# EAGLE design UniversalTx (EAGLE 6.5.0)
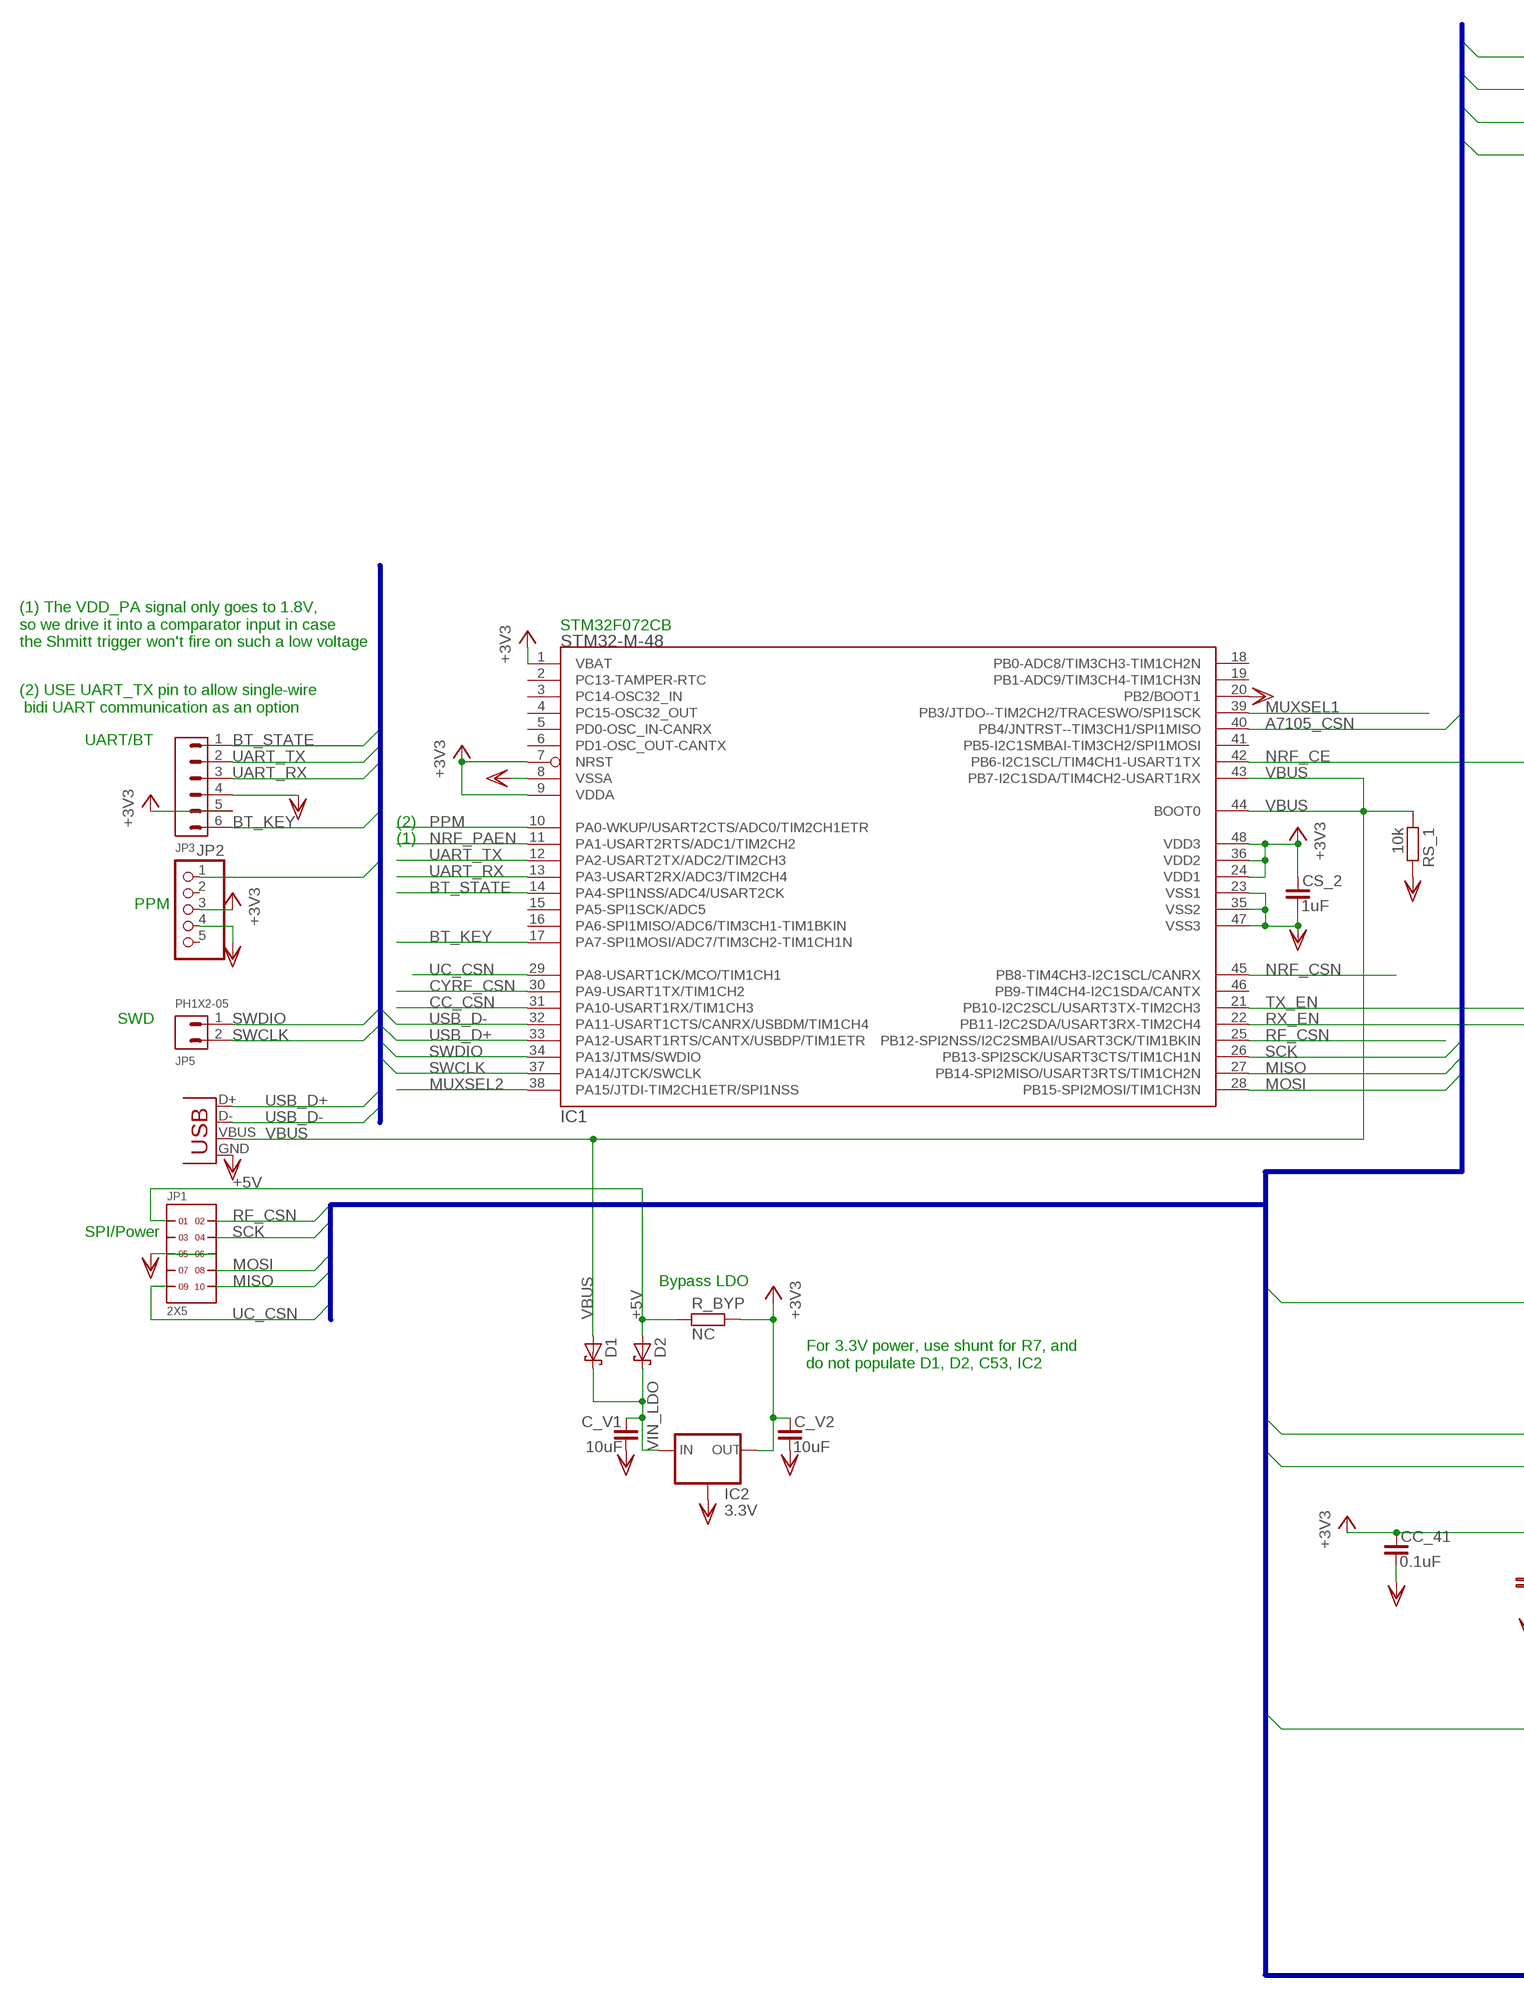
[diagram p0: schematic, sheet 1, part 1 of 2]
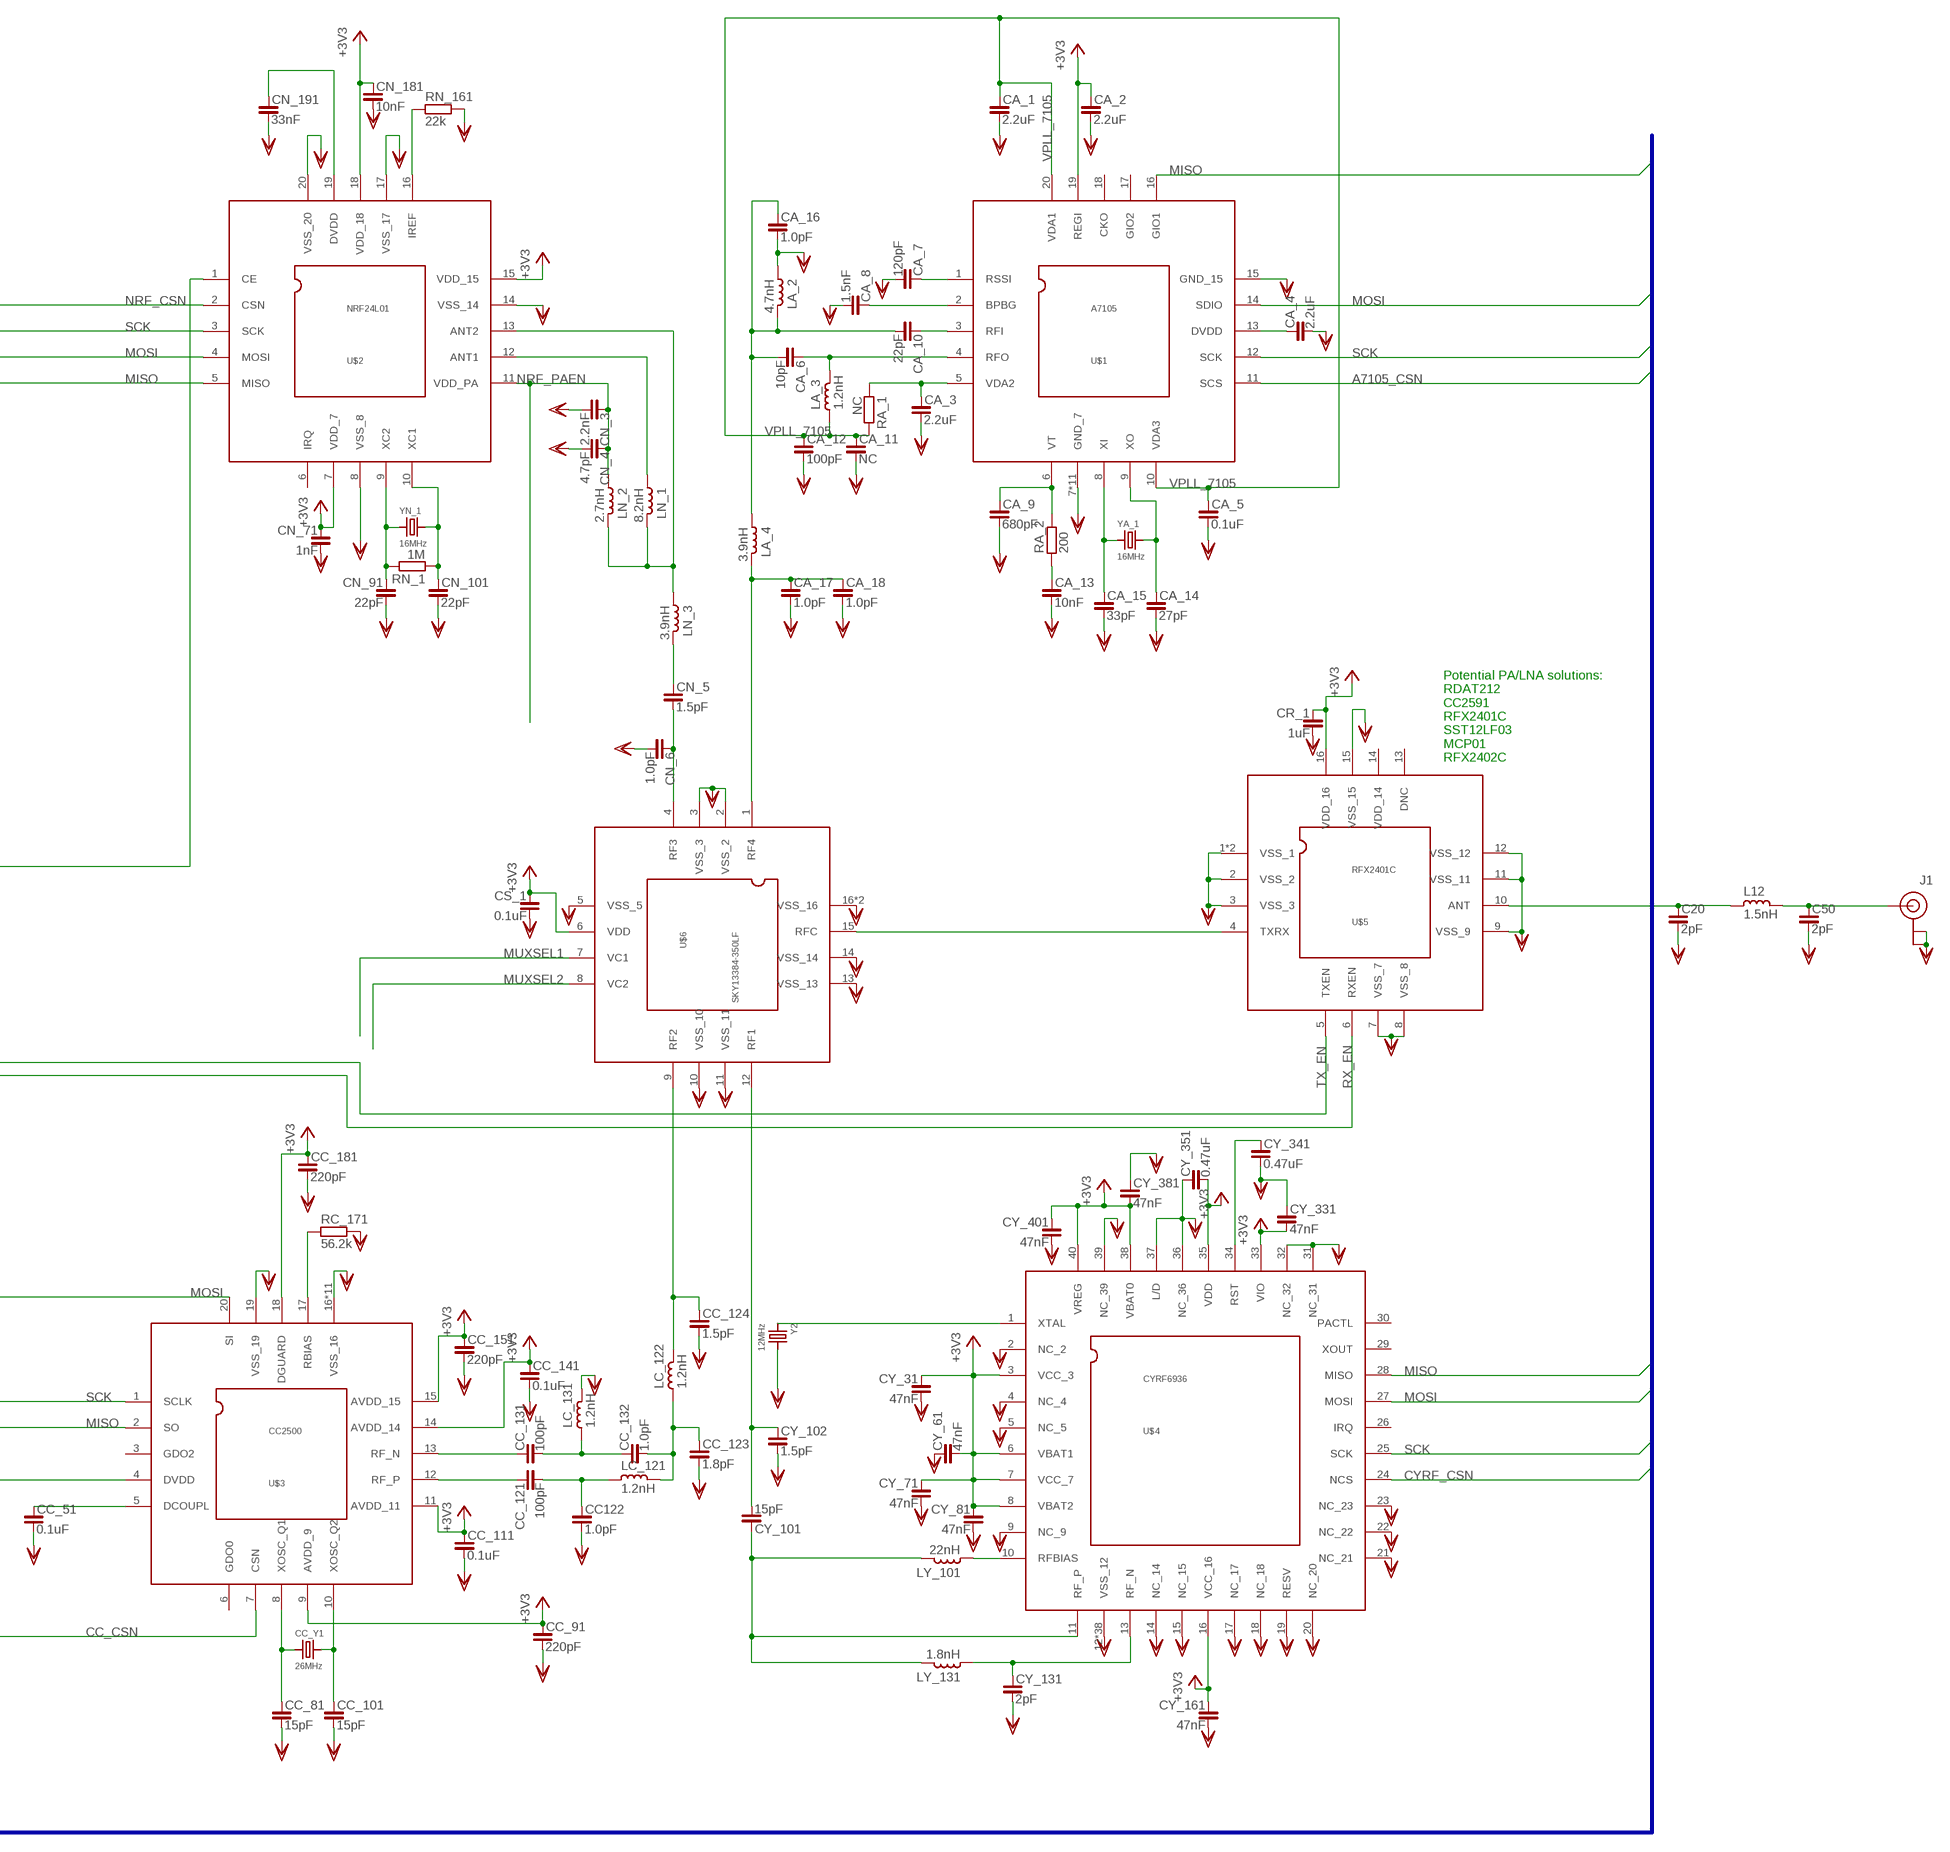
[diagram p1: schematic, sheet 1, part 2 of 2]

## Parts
C20  2pF  C_0402  [C0402]
C50  2pF  C_0402  [C0402]
C_V1  10uF  C_0805  [C0805]
C_V2  10uF  C_0805  [C0805]
CA_1  2.2uF  C_0402  [C0402]
CA_2  2.2uF  C_0402  [C0402]
CA_3  2.2uF  C_0402  [C0402]
CA_4  2.2uF  C_0402  [C0402]
CA_5  0.1uF  C_0402  [C0402]
CA_6  10pF  C_0402  [C0402]
CA_7  120pF  C_0402  [C0402]
CA_8  1.5nF  C_0402  [C0402]
CA_9  680pF  C_0402  [C0402]
CA_10  22pF  C_0402  [C0402]
CA_11  NC  C_0402  [C0402]
CA_12  100pF  C_0402  [C0402]
CA_13  10nF  C_0402  [C0402]
CA_14  27pF  C_0402  [C0402]
CA_15  33pF  C_0402  [C0402]
CA_16  1.0pF  C_0402  [C0402]
CA_17  1.0pF  C_0402  [C0402]
CA_18  1.0pF  C_0402  [C0402]
CC122  1.0pF  C_0402  [C0402]
CC_41  0.1uF  C_0402  [C0402]
CC_51  0.1uF  C_0402  [C0402]
CC_81  15pF  C_0402  [C0402]
CC_91  220pF  C_0402  [C0402]
CC_101  15pF  C_0402  [C0402]
CC_111  0.1uF  C_0402  [C0402]
CC_121  100pF  C_0402  [C0402]
CC_123  1.8pF  C_0402  [C0402]
CC_124  1.5pF  C_0402  [C0402]
CC_131  100pF  C_0402  [C0402]
CC_132  1.0pF  C_0402  [C0402]
CC_141  0.1uF  C_0402  [C0402]
CC_151  220pF  C_0402  [C0402]
CC_181  220pF  C_0402  [C0402]
CC_Y1  26MHz  CRYSTAL.3.2X2.5MM  [3.2X2.5MM]
CN_3  2.2nF  C_0402  [C0402]
CN_4  4.7pF  C_0402  [C0402]
CN_5  1.5pF  C_0402  [C0402]
CN_6  1.0pF  C_0402  [C0402]
CN_71  1nF  C_0402  [C0402]
CN_91  22pF  C_0402  [C0402]
CN_101  22pF  C_0402  [C0402]
CN_181  10nF  C_0402  [C0402]
CN_191  33nF  C_0402  [C0402]
CR_1  1uF  C_0402  [C0402]
CS_1  0.1uF  C_0402  [C0402]
CS_2  1uF  C_0402  [C0402]
CY_31  47nF  C_0402  [C0402]
CY_61  47nF  C_0402  [C0402]
CY_71  47nF  C_0402  [C0402]
CY_81  47nF  C_0402  [C0402]
CY_101  15pF  C_0402  [C0402]
CY_102  1.5pF  C_0402  [C0402]
CY_131  2pF  C_0402  [C0402]
CY_161  47nF  C_0402  [C0402]
CY_331  47nF  C_0402  [C0402]
CY_341  0.47uF  C_0402  [C0402]
CY_351  0.47uF  C_0402  [C0402]
CY_381  47nF  C_0402  [C0402]
CY_401  47nF  C_0402  [C0402]
D1  LSM115J  [DO214BA]
D2  LSM115J  [DO214BA]
IC1  STM32-M-48  [LQFP48]
IC2  3.3V  LD1117SOT223  [SOT223]
J1  U.FL  [U.FL]
JP1  2X5  [2X5]
JP2  PINHD-1X05_2.54-S  [1X05-S]
JP3  PH1X6-05  [PH005-1-6]
JP5  PH1X2-05  [PH005-1-2]
JP6  USBSMD  [USB-MINIB]
L12  1.5nH  L_0402  [L0402]
LA_2  4.7nH  L_0402  [L0402]
LA_3  1.2nH  L_0402  [L0402]
LA_4  3.9nH  L_0402  [L0402]
LC_121  1.2nH  L_0402  [L0402]
LC_122  1.2nH  L_0402  [L0402]
LC_131  1.2nH  L_0402  [L0402]
LN_1  8.2nH  L_0402  [L0402]
LN_2  2.7nH  L_0402  [L0402]
LN_3  3.9nH  L_0402  [L0402]
LY_101  22nH  L_0402  [L0402]
LY_131  1.8nH  L_0402  [L0402]
R_BYP  NC  R_0805  [R0805]
RA_1  NC  R_0402  [R0402]
RA_2  200  R_0402  [R0402]
RC_171  56.2k  R_0402  [R0402]
RN_1  1M  R_0402  [R0402]
RN_161  22k  R_0402  [R0402]
RS_1  10k  R_0402  [R0402]
U$1  A7105  [QFN20-4X4-PAD]
U$2  NRF24L01  [QFN20-4X4-NRF]
U$3  CC2500  [QFN20-4X4-PAD]
U$4  CYRF6936  [QFN40-6X6]
U$5  RFX2401C  [QFN16-3X3-PAD]
U$6  SKY13384-350LF  [QFN16-3X3-PAD]
Y2  12MHz  CRYSTAL.3.2X2.5MM  [3.2X2.5MM]
YA_1  16MHz  CRYSTAL.3.2X2.5MM  [3.2X2.5MM]
YN_1  16MHz  CRYSTAL.3.2X2.5MM  [3.2X2.5MM]

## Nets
+3V3: C_V2.1 CA_2.1 CC_41.1 CC_91.1 CC_111.1 CC_141.1 CC_151.1 CC_181.1 CN_71.1 CN_181.1 CR_1.1 CS_1.1 CS_2.1 CY_31.1 CY_61.2 CY_71.1 CY_81.1 CY_161.1 CY_331.2 CY_351.2 CY_381.2 CY_401.1 IC1.1(VBAT) IC1.7(NRST) IC1.9(VDDA) IC1.24(VDD1) IC1.36(VDD2) IC1.48(VDD3) IC2.2(OUT) JP2.3 JP3.5 R_BYP.2 U$1.19(REGI) U$2.7(VDD_7) U$2.15(VDD_15) U$2.18(VDD_18) U$3.4(DVDD) U$3.9(AVDD_9) U$3.11(AVDD_11) U$3.14(AVDD_14) U$3.15(AVDD_15) U$3.18(DGUARD) U$4.3(VCC_3) U$4.6(VBAT1) U$4.7(VCC_7) U$4.8(VBAT2) U$4.16(VCC_16) U$4.33(VIO) U$4.35(VDD) U$4.38(VBAT0) U$4.40(VREG) U$5.16(VDD_16) U$6.6(VDD)
+5V: D2.A JP1.1 R_BYP.1
A7105_CSN: IC1.40(PB4/JNTRST--TIM3CH1/SPI1MISO) U$1.11(SCS)
BT_KEY: IC1.17(PA7-SPI1MOSI/ADC7/TIM3CH2-TIM1CH1N) JP3.6
BT_STATE: IC1.14(PA4-SPI1NSS/ADC4/USART2CK) JP3.1
CC_CSN: IC1.31(PA10-USART1RX/TIM1CH3) U$3.7(CSN)
CYRF_CSN: IC1.30(PA9-USART1TX/TIM1CH2) U$4.24(NCS)
MISO: IC1.27(PB14-SPI2MISO/USART3RTS/TIM1CH2N) JP1.10 U$1.16(GIO1) U$2.5(MISO) U$3.2(SO) U$4.28(MISO)
MOSI: IC1.28(PB15-SPI2MOSI/TIM1CH3N) JP1.8 U$1.14(SDIO) U$2.4(MOSI) U$3.20(SI) U$4.27(MOSI)
MUXSEL1: IC1.39(PB3/JTDO--TIM2CH2/TRACESWO/SPI1SCK) U$6.7(VC1)
MUXSEL2: IC1.38(PA15/JTDI-TIM2CH1ETR/SPI1NSS) U$6.8(VC2)
N$1: CN_101.1 RN_1.1 U$2.10(XC1) YN_1.3
N$2: CN_91.1 RN_1.2 U$2.9(XC2) YN_1.1
N$3: CN_191.1 U$2.19(DVDD)
N$4: CA_9.1 RA_2.2 U$1.6(VT)
N$5: LN_1.1 LN_2.1 LN_3.2 U$2.13(ANT2)
N$7: C50.1 J1.P$3(SIGNAL) L12.1
N$8: CN_5.1 LN_3.1
N$9: CN_5.2 CN_6.1 U$6.4(RF3)
N$10: RN_161.1 U$2.16(IREF)
N$11: CA_13.1 RA_2.1
N$12: CA_14.1 U$1.9(XO) YA_1.3
N$14: CC_131.1 U$3.13(RF_N)
N$15: LN_1.2 U$2.12(ANT1)
N$16: CC_121.1 U$3.12(RF_P)
N$17: CA_15.1 U$1.8(XI) YA_1.1
N$18: CA_4.1 U$1.13(DVDD)
N$24: CC_123.1 CC_132.2 LC_121.1 LC_122.2
N$25: CA_17.1 CA_18.1 LA_4.1 U$6.1(RF4)
N$26: CA_7.1 U$1.1(RSSI)
N$27: CA_8.1 U$1.2(BPBG)
N$28: CA_10.1 U$1.3(RFI)
N$29: CA_6.1 LA_3.1 U$1.4(RFO)
N$30: CA_3.1 RA_1.1 U$1.5(VDA2)
N$31: C20.1 L12.2 U$5.10(ANT)
N$32: CC_51.1 U$3.5(DCOUPL)
N$37: RC_171.1 U$3.17(RBIAS)
N$38: CC_101.1 CC_Y1.3 U$3.10(XOSC_Q2)
N$39: CC_81.1 CC_Y1.1 U$3.8(XOSC_Q1)
N$40: CC122.1 CC_121.2 LC_121.2
N$41: CC_131.2 CC_132.1 LC_131.2
N$42: U$5.4(TXRX) U$6.15(RFC)
N$43: CY_341.1 U$4.34(RST)
N$44: U$4.1(XTAL) Y2.1
N$45: LY_101.2 U$4.10(RFBIAS)
N$46: CY_101.1 LY_101.1 LY_131.1 U$4.11(RF_P)
N$47: CY_131.1 LY_131.2 U$4.13(RF_N)
N$48: CA_6.2 CA_10.2 CA_16.1 LA_2.1 LA_4.2
N$49: CY_101.2 CY_102.1 U$6.12(RF1)
N$50: CC_124.1 LC_122.1 U$6.9(RF2)
NRF_CE: IC1.42(PB6-I2C1SCL/TIM4CH1-USART1TX) U$2.1(CE)
NRF_CSN: IC1.45(PB8-TIM4CH3-I2C1SCL/CANRX) U$2.2(CSN)
NRF_PAEN: CN_3.1 CN_4.1 IC1.11(PA1-USART2RTS/ADC1/TIM2CH2) LN_2.2 U$2.11(VDD_PA)
PPM: IC1.10(PA0-WKUP/USART2CTS/ADC0/TIM2CH1ETR) JP2.1
RF_CSN: IC1.25(PB12-SPI2NSS/I2C2SMBAI/USART3CK/TIM1BKIN) JP1.2
RX_EN: IC1.22(PB11-I2C2SDA/USART3RX-TIM2CH4) U$5.6(RXEN)
SCK: IC1.26(PB13-SPI2SCK/USART3CTS/TIM1CH1N) JP1.4 U$1.12(SCK) U$2.3(SCK) U$3.1(SCLK) U$4.25(SCK)
SWCLK: IC1.37(PA14/JTCK/SWCLK) JP5.2
SWDIO: IC1.34(PA13/JTMS/SWDIO) JP5.1
TX_EN: IC1.21(PB10-I2C2SCL/USART3TX-TIM2CH3) U$5.5(TXEN)
UART_RX: IC1.13(PA3-USART2RX/ADC3/TIM2CH4) JP3.3
UART_TX: IC1.12(PA2-USART2TX/ADC2/TIM2CH3) JP3.2
UC_CSN: IC1.29(PA8-USART1CK/MCO/TIM1CH1) JP1.9
USB_D+: IC1.33(PA12-USART1RTS/CANTX/USBDP/TIM1ETR) JP6.D+
USB_D-: IC1.32(PA11-USART1CTS/CANRX/USBDM/TIM1CH4) JP6.D-
VBUS: D1.A IC1.43(PB7-I2C1SDA/TIM4CH2-USART1RX) IC1.44(BOOT0) JP6.VBUS RS_1.1
VIN_LDO: C_V1.1 D1.C D2.C IC2.3(IN)
VPLL_7105: CA_1.1 CA_5.1 CA_11.1 CA_12.1 LA_3.2 RA_1.2 U$1.10(VDA3) U$1.20(VDA1)
VSS: C20.2 C50.2 C_V1.2 C_V2.2 CA_1.2 CA_2.2 CA_3.2 CA_4.2 CA_5.2 CA_7.2 CA_8.2 CA_9.2 CA_11.2 CA_12.2 CA_13.2 CA_14.2 CA_15.2 CA_16.2 CA_17.2 CA_18.2 CC122.2 CC_41.2 CC_51.2 CC_81.2 CC_91.2 CC_101.2 CC_111.2 CC_123.2 CC_124.2 CC_141.2 CC_151.2 CC_181.2 CN_3.2 CN_4.2 CN_6.2 CN_71.2 CN_91.2 CN_101.2 CN_181.2 CN_191.2 CR_1.2 CS_1.2 CS_2.2 CY_31.2 CY_61.1 CY_71.2 CY_81.2 CY_102.2 CY_131.2 CY_161.2 CY_331.1 CY_341.2 CY_351.1 CY_381.1 CY_401.2 IC1.8(VSSA) IC1.20(PB2/BOOT1) IC1.23(VSS1) IC1.35(VSS2) IC1.47(VSS3) IC2.1(GND) IC2.4(GND) J1.P$1(GND) J1.P$2(GND) JP1.5 JP1.6 JP2.4 JP3.4 JP6.GND LA_2.2 LC_131.1 RC_171.2 RN_161.2 RS_1.2 U$1.7(GND_7) U$1.15(GND_15) U$1.21(GND_7) U$1.P$1(GND_7) U$1.P$2(GND_7) U$1.P$3(GND_7) U$1.P$4(GND_7) U$1.P$5(GND_7) U$1.P$6(GND_7) U$1.P$7(GND_7) U$1.P$8(GND_7) U$1.P$9(GND_7) U$2.8(VSS_8) U$2.14(VSS_14) U$2.17(VSS_17) U$2.20(VSS_20) U$3.16(VSS_16) U$3.19(VSS_19) U$3.21(VSS_16) U$3.P$1(VSS_16) U$3.P$2(VSS_16) U$3.P$3(VSS_16) U$3.P$4(VSS_16) U$3.P$5(VSS_16) U$3.P$6(VSS_16) U$3.P$7(VSS_16) U$3.P$8(VSS_16) U$3.P$9(VSS_16) U$4.2(NC_2) U$4.4(NC_4) U$4.5(NC_5) U$4.9(NC_9) U$4.12(VSS_12) U$4.14(NC_14) U$4.15(NC_15) U$4.17(NC_17) U$4.18(NC_18) U$4.19(RESV) U$4.20(NC_20) U$4.21(NC_21) U$4.22(NC_22) U$4.23(NC_23) U$4.31(NC_31) U$4.32(NC_32) U$4.36(NC_36) U$4.37(L/D) U$4.39(NC_39) U$4.P$1(VSS_12) U$4.P$2(VSS_12) U$4.P$3(VSS_12) U$4.P$4(VSS_12) U$4.P$5(VSS_12) U$4.P$6(VSS_12) U$4.P$7(VSS_12) U$4.P$8(VSS_12) U$4.P$9(VSS_12) U$4.P$10(VSS_12) U$4.P$11(VSS_12) U$4.P$12(VSS_12) U$4.P$13(VSS_12) U$4.P$14(VSS_12) U$4.P$15(VSS_12) U$4.P$16(VSS_12) U$4.P$17(VSS_12) U$4.P$18(VSS_12) U$4.P$19(VSS_12) U$4.P$20(VSS_12) U$4.P$21(VSS_12) U$4.P$22(VSS_12) U$4.P$23(VSS_12) U$4.P$24(VSS_12) U$4.P$25(VSS_12) U$4.P$26(VSS_12) U$4.P$27(VSS_12) U$4.P$28(VSS_12) U$4.P$29(VSS_12) U$4.P$30(VSS_12) U$4.P$31(VSS_12) U$4.P$32(VSS_12) U$4.P$33(VSS_12) U$4.P$34(VSS_12) U$4.P$35(VSS_12) U$4.P$36(VSS_12) U$4.P$37(VSS_12) U$5.1(VSS_1) U$5.2(VSS_2) U$5.3(VSS_3) U$5.7(VSS_7) U$5.8(VSS_8) U$5.9(VSS_9) U$5.11(VSS_11) U$5.12(VSS_12) U$5.15(VSS_15) U$5.17(VSS_1) U$6.2(VSS_2) U$6.3(VSS_3) U$6.5(VSS_5) U$6.10(VSS_10) U$6.11(VSS_11) U$6.13(VSS_13) U$6.14(VSS_14) U$6.16(VSS_16) U$6.17(VSS_16) Y2.3
Unconnected: IC1.2(PC13-TAMPER-RTC) IC1.3(PC14-OSC32_IN) IC1.4(PC15-OSC32_OUT) IC1.5(PD0-OSC_IN-CANRX) IC1.6(PD1-OSC_OUT-CANTX) IC1.15(PA5-SPI1SCK/ADC5) IC1.16(PA6-SPI1MISO/ADC6/TIM3CH1-TIM1BKIN) IC1.18(PB0-ADC8/TIM3CH3-TIM1CH2N) IC1.19(PB1-ADC9/TIM3CH4-TIM1CH3N) IC1.41(PB5-I2C1SMBAI-TIM3CH2/SPI1MOSI) IC1.46(PB9-TIM4CH4-I2C1SDA/CANTX) JP1.3 JP1.7 JP2.2 JP2.5 U$1.17(GIO2) U$1.18(CKO) U$2.6(IRQ) U$3.3(GDO2) U$3.6(GDO0) U$4.26(IRQ) U$4.29(XOUT) U$4.30(PACTL) U$5.13(DNC) U$5.14(VDD_14)

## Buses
SCK,MOSI,MISO,NRF_CSN,CC_CSN,A7105_CSN,CYRF_CSN,UC_CSN,RF_CSN
PPM,UART_TX,UART_RX,BT_KEY,BT_STATE,USB_D+,USB_D-,SWDIO,SWCLK,NRF_PAEN

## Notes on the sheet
- STM32F072CB
- Potential PA/LNA solutions:
  RDAT212
  CC2591
  RFX2401C
  SST12LF03
  MCP01
  RFX2402C
- (1) The VDD_PA signal only goes to 1.8V,
  so we drive it into a comparator input in case
  the Shmitt trigger won't fire on such a low voltage
- (2) USE UART_TX pin to allow single-wire
   bidi UART communication as an option
- UART/BT
- (2)
- (1)
- PPM
- SWD
- SPI/Power
- Bypass LDO
- For 3.3V power, use shunt for R7, and
  do not populate D1, D2, C53, IC2

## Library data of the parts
C20 C50 CY_131 = rc-master-smd:C_: NON-POLARIZED CAP; DIGIKEY#: 490-6226-1-ND; MANF: Murata; MANF#: GRM1555C1H2R0BA01D; MOUSER#: 81-GRM1555C1H2R0BA1D
C_V1 C_V2 = rc-master-smd:C_: NON-POLARIZED CAP; DIGIKEY#: 490-1709-1-ND; MANF: Murata; MANF#: GRM21BR61A106KE19L; MOUSER#: 81-GRM21BR61A106KE19
CA_1-CA_4 = rc-master-smd:C_: NON-POLARIZED CAP; DIGIKEY#: 399-7375-1-ND; MANF: Kemet; MANF#: C0402C225M8PACTU; MOUSER#: 80-C0402C225M8P
CA_5 CC_41 CC_51 CC_111 CC_141 CS_1 = rc-master-smd:C_: NON-POLARIZED CAP; DIGIKEY#: 490-1318-1-ND; MANF: Murata; MANF#: GRM155R61A104KA01D; MOUSER#: 81-GRM155R61A104KA1D
CA_6 = rc-master-smd:C_: NON-POLARIZED CAP; DIGIKEY#: 490-6186-1-ND; MANF: Murata; MANF#: GRM1555C1H100FA01D; MOUSER#: 81-GRM1555C1H100FA1D
CA_7 = rc-master-smd:C_: NON-POLARIZED CAP; DIGIKEY#: 490-8183-1-ND; MANF: Murata; MANF#: GRM1555C1H121GA01D; MOUSER#: 81-GRM1555C1H121GA1D
CA_8 = rc-master-smd:C_: NON-POLARIZED CAP; DIGIKEY#: 490-6354-1-ND; MANF: Murata; MANF#: GRM155R71H152KA01J; MOUSER#: 81-GRM155R71H152KA1J
CA_9 = rc-master-smd:C_: NON-POLARIZED CAP; DIGIKEY#: 490-3240-1-ND; MANF: Murata; MANF#: GRM1555C1H681JA01D; MOUSER#: 81-GRM1555C1H681JA1D
CA_10 CN_91 CN_101 = rc-master-smd:C_: NON-POLARIZED CAP; DIGIKEY#: 490-8173-1-ND; MANF: Murata; MANF#: GRM1555C1E220GA01D; MOUSER#: 81-GRM1555C1E220GA1D
CA_11 = rc-master-smd:C_: NON-POLARIZED CAP
CA_12 CC_121 CC_131 = rc-master-smd:C_: NON-POLARIZED CAP; DIGIKEY#: 490-6188-1-ND; MANF: Murata; MANF#: GRM1555C1H101GA01D; MOUSER#: 81-GRM1555C1H101GA1D
CA_13 CN_181 = rc-master-smd:C_: NON-POLARIZED CAP; DIGIKEY#: 490-1313-1-ND; MANF: Murata; MANF#: GRM155R71C103KA01D; MOUSER#: 81-GRM155R71C103KA1D
CA_14 = rc-master-smd:C_: NON-POLARIZED CAP; DIGIKEY#: 490-6224-1-ND; MANF: Murata; MANF#: GRM1555C1H270GA01D; MOUSER#: 81-GRM1555C1H270GA1D
CA_15 = rc-master-smd:C_: NON-POLARIZED CAP; DIGIKEY#: 490-6232-1-ND; MANF: Murata; MANF#: GRM1555C1H330GA01D; MOUSER#: 81-GRM1555C1H330GA1D
CA_16-CA_18 CC122 CC_132 CN_6 = rc-master-smd:C_: NON-POLARIZED CAP; DIGIKEY#: 490-6206-1-ND; MANF: Murata; MANF#: GRM1555C1H1R0BA01D; MOUSER#: 81-GRM1555C1H1R0BA1D
CC_81 CC_101 CY_101 = rc-master-smd:C_: NON-POLARIZED CAP; DIGIKEY#: 490-6200-1-ND; MANF: Murata; MANF#: GRM1555C1H150FA01D; MOUSER#: 81-GRM1555C1H150FA1D
CC_91 CC_151 CC_181 = rc-master-smd:C_: NON-POLARIZED CAP; DIGIKEY#: 490-1293-1-ND; MANF: Murata; MANF#: GRM1555C1H221JA01D; MOUSER#: 81-GRM1555C1H221JA1D
CC_123 = rc-master-smd:C_: NON-POLARIZED CAP; DIGIKEY#: 490-6215-1-ND; MANF: Murata; MANF#: GRM1555C1H1R8BA01D; MOUSER#: 81-GRM1555C1H1R8BA1D
CC_124 CN_5 CY_102 = rc-master-smd:C_: NON-POLARIZED CAP; DIGIKEY#: 490-6212-1-ND; MANF: Murata; MANF#: GRM1555C1H1R5BA01D; MOUSER#: 81-GRM1555C1H1R5BA1D
CC_Y1 = UniversalTx:CRYSTAL; DIGIKEY#: 887-1716-1-ND; MANF: TXC; MANF#: AB-26.000MAGE-T; MOUSER#: 717-AB-26.000MAGE-T
CN_3 = rc-master-smd:C_: NON-POLARIZED CAP; DIGIKEY#: 490-6358-1-ND; MANF: Murata; MANF#: GRM155R71H222JA01D; MOUSER#: 81-GRM155R71H222JA1D
CN_4 = rc-master-smd:C_: NON-POLARIZED CAP; DIGIKEY#: 490-6244-1-ND; MANF: Murata; MANF#: GRM1555C1H4R7BA01D; MOUSER#: 81-GRM1555C1H4R7BA1D
CN_71 = rc-master-smd:C_: NON-POLARIZED CAP; DIGIKEY#: 490-3244-1-ND; MANF: Murata; MANF#: GRM1555C1H102JA01D; MOUSER#: 81-GRM1555C1H102JA1D
CN_191 = rc-master-smd:C_: NON-POLARIZED CAP; DIGIKEY#: 490-6333-1-ND; MANF: Murata; MANF#: GRM155R71C333KA01J; MOUSER#: 81-GRM155R71C333KA1J
CR_1 CS_2 = rc-master-smd:C_: NON-POLARIZED CAP; DIGIKEY#: 490-3890-1-ND; MANF: Murata; MANF#: GRM155R61A105KE15D; MOUSER#: 81-GRM155R61A105KE15
CY_31 CY_61 CY_71 CY_81 CY_161 CY_331 CY_381 CY_401 = rc-master-smd:C_: NON-POLARIZED CAP; DIGIKEY#: 490-6313-1-ND; MANF: Murata; MANF#: GRM155R61C473KA01D; MOUSER#: 81-GRM155R61C473KA1D
CY_341 CY_351 = rc-master-smd:C_: NON-POLARIZED CAP; DIGIKEY#: 490-3266-1-ND; MANF: Murata; MANF#: GRM155R60J474KE19D; MOUSER#: 81-GRM155R60J474KE9D
D1 D2 = UniversalTx:LSM115J; DIGIKEY#: LSM115JE3/TR13CT-ND; MANF: Microsemi; MANF#: LSM115JE3/TR13
IC1 = UniversalTx:STM32-M-48: STM32F103 Medium Density 48pins; DIGIKEY#: 497-14645-ND; MANF: STMicroelectronics; MANF#: STM32F072CBT6
IC2 = UniversalTx:LD1117: Voltage Regulator LM1117 Standard adjustable voltage regulator but in SMD form. Spark Fun Electronics SKU : COM-00595; DIGIKEY#: 497-1241-1-ND; MANF: STMicroelectronics; MANF#: LD1117S33CTR; MOUSER#: 511-LD1117S33C
J1 = UniversalTx:U.FL: SMD antenna connector- WRL-09144; DIGIKEY#: WM5587CT-ND; MANF: Molex; MANF#: 0734120110; PROD_ID: CONN-09193
JP1 = UniversalTx:2X5
JP2 = UniversalTx:PINHD-1X05: PIN HEADER
JP3 = UniversalTx:PH1X6
JP5 = UniversalTx:PH1X2
JP6 = UniversalTx:USB: USB Connectors USB-B-PTH is fully proven SKU : PRT-00139/CONN-08278 USB-miniB is fully proven SKU : PRT-00587 USB-A-PCB is untested. USB-A-H is throughly reviewed, but untested. Spark Fun Electronics SKU : PRT-00437 USB-B-SMT is throughly reviewed, but untested. Needs silkscreen touching up.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; DIGIKEY#: 670-1190-1-ND; MANF: JAE; MANF#: DX2R005HN2E700; PROD_ID: CONN-08193
L12 = rc-master-smd:L_: INDUCTOR; DIGIKEY#: PCD1900CT-ND; MANF: Panasonic; MANF#: ELJ-RF1N5ZFB; MOUSER#: 667-ELJ-RF1N5ZFB
LA_2 = rc-master-smd:L_: INDUCTOR; DIGIKEY#: PCD1906CT-ND; MANF: Panasonic; MANF#: ELJ-RF4N7ZFB; MOUSER#: 667-ELJ-RF4N7ZFB
LA_3 LC_121 LC_122 LC_131 = rc-master-smd:L_: INDUCTOR; DIGIKEY#: PCD1899CT-ND; MANF: Panasonic; MANF#: ELJ-RF1N2ZFB; MOUSER#: 667-ELJ-RF1N2ZFB
LA_4 LN_3 = rc-master-smd:L_: INDUCTOR; DIGIKEY#: PCD1905CT-ND; MANF: Panasonic; MANF#: ELJ-RF3N9ZFB; MOUSER#: 667-ELJ-RF3N9ZFB
LN_1 = rc-master-smd:L_: INDUCTOR; DIGIKEY#: PCD1909CT-ND; MANF: Panasonic; MANF#: ELJ-RF8N2ZFB; MOUSER#: 667-ELJ-RF8N2ZFB
LN_2 = rc-master-smd:L_: INDUCTOR; DIGIKEY#: PCD1903CT-ND; MANF: Panasonic; MANF#: ELJ-RF2N7ZFB; MOUSER#: 667-ELJ-RF2N7ZFB
LY_101 = rc-master-smd:L_: INDUCTOR; DIGIKEY#: PCD1914CT-ND; MANF: Panasonic; MANF#: ELJ-RF22NGFB; MOUSER#: 667-ELJ-RF22NGFB
LY_131 = rc-master-smd:L_: INDUCTOR; DIGIKEY#: PCD1901CT-ND; MANF: Panasonic; MANF#: ELJ-RF1N8ZFB; MOUSER#: 667-ELJ-RF1N8ZFB
R_BYP RA_1 = rc-master-smd:R_: RESISTOR
RA_2 = rc-master-smd:R_: RESISTOR; DIGIKEY#: P200JCT-ND; MANF: Panasonic; MANF#: ERJ-2GEJ201X; MOUSER#: 667-ERJ-2GEJ201X
RC_171 = rc-master-smd:R_: RESISTOR; DIGIKEY#: P56.2KLCT-ND; MANF: Panasonic; MANF#: ERJ-2RKF5622X; MOUSER#: 667-ERJ-2RKF5622X
RN_1 = rc-master-smd:R_: RESISTOR; DIGIKEY#: P1.0MJCT-ND; MANF: Panasonic; MANF#: ERJ-2GEJ105X; MOUSER#: 667-ERJ-2GEJ105X
RN_161 = rc-master-smd:R_: RESISTOR; DIGIKEY#: P22KJCT-ND; MANF: Panasonic; MANF#: ERJ-2GEJ223X; MOUSER#: 667-ERJ-2GEJ223X
RS_1 = rc-master-smd:R_: RESISTOR; DIGIKEY#: P10KACT-ND; MANF: Panasonic; MANF#: ERJ-6GEYJ103V; MOUSER#: 667-ERJ-6GEYJ103V
U$1 = UniversalTx:A7105; MANF: Amiccom
U$2 = UniversalTx:NRF24L01: nRF24L01 Single chip 2.4GHz transceiver from Nordic Semiconductors.; DIGIKEY#: 1490-1033-1-ND; MANF: Nordic; MANF#: NRF24L01P-R7
U$3 = UniversalTx:CC2500; DIGIKEY#: 296-19586-2-ND; MANF: TI; MANF#: CC2500RTKR
U$4 = UniversalTx:CYRF6936; DIGIKEY#: 428-2962-ND; MANF: Cypress; MANF#: CYRF6936-40LTXC
U$5 = UniversalTx:RFX2401C; MANF: RF Axis; MANF#: RFX2401C
U$6 = UniversalTx:SKY13384-350LF; DIGIKEY#: 863-1456-1-ND; MANF: Skyworks; MANF#: SKY13384-350LF
Y2 = UniversalTx:CRYSTAL; DIGIKEY#: 887-1701-1-ND; MANF: TXC; MANF#: AB-12.000MALE-T; MOUSER#: 717-AB-12.000MALE-T
YA_1 YN_1 = UniversalTx:CRYSTAL; DIGIKEY#: 887-1707-1-ND; MANF: TXC; MANF#: AB-16.000MAGE-T; MOUSER#: 717-AB-16.000MAGE-T

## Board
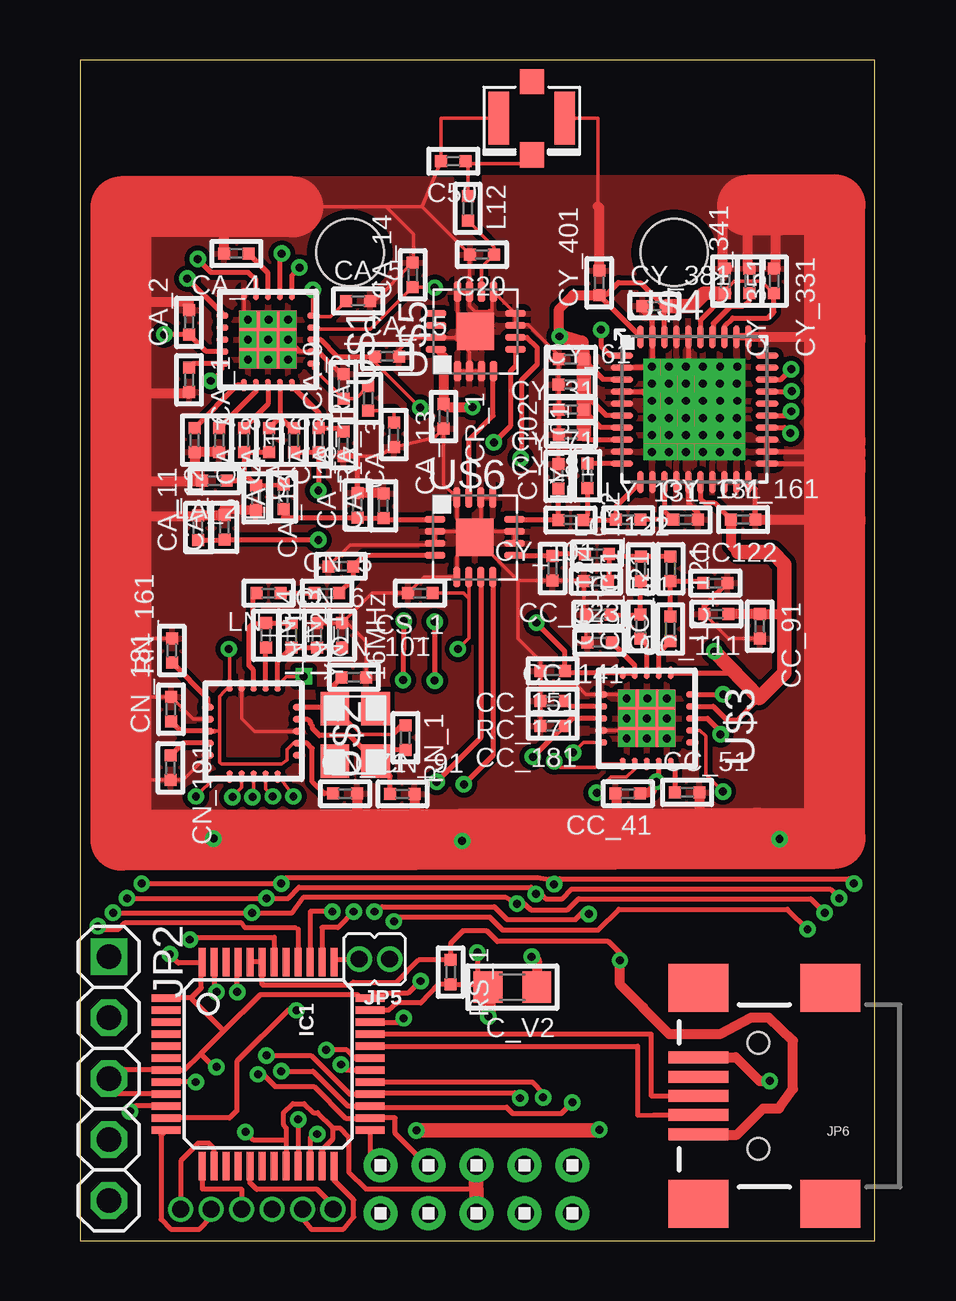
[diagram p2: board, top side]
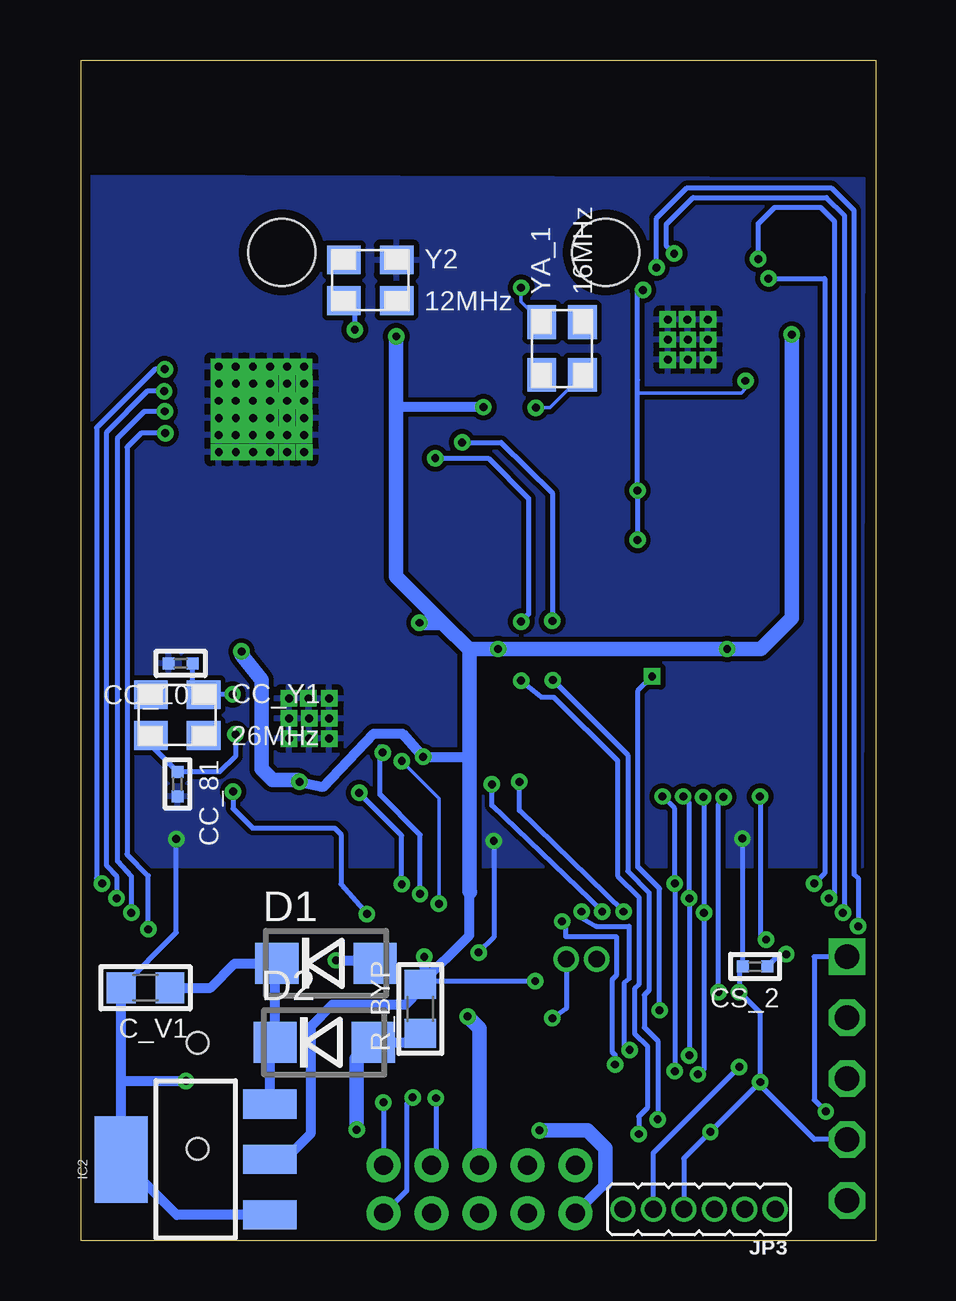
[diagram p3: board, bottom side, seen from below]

Size 33.12 x 49.22 mm. Coordinates in mm from the lower left corner, seen from the top.
Outline: 0,0 33.12,0 33.12,49.22 0,49.22 0,0
Copper layers (1*16): Top 0.0356mm / dielectric 1.5011mm / Bottom 0.0356mm
Design rules "LaenPCBOrder *": minimum track width 6mil, minimum drill 13mil, track to track 8mil, track to pad 6mil, pad to pad 6mil, via to via 6mil, smd to smd 6mil, copper to edge 15mil, drill to drill 6mil, minimum pad ring 7mil, minimum via ring 7mil, stop-mask expansion 3mil, vias tented up to drill 0mil, thermal gap 10mil
Holes 2.8 mm at 11.25,41.2 24.77,41.2

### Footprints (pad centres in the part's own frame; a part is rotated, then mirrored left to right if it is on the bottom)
C0402 = smd 0.5 x 0.5: 1 -0.508,0; 2 0.508,0
C0805 = smd 1.2 x 1.3: 1 -1.016,0; 2 1.016,0
3.2X2.5MM = smd 1.4 x 1.2: 1 -1.1,-0.85; 2 1.1,-0.85; 3 1.1,0.85; 4 -1.1,0.85
DO214BA = smd 1.8 x 1.7: A 2.05,0; C -2.05,0
LQFP48 = smd 0.3 x 1.2: 1 -2.75,-4.25; 2 -2.25,-4.25; 3 -1.75,-4.25; 4 -1.25,-4.25; 5 -0.75,-4.25; 6 -0.25,-4.25; 7 0.25,-4.25; 8 0.75,-4.25; 9 1.25,-4.25; 10 1.75,-4.25; 11 2.25,-4.25; 12 2.75,-4.25; 25 2.75,4.25; 26 2.25,4.25; 27 1.75,4.25; 28 1.25,4.25; 29 0.75,4.25; 30 0.25,4.25; 31 -0.25,4.25; 32 -0.75,4.25; 33 -1.25,4.25; 34 -1.75,4.25; 35 -2.25,4.25; 36 -2.75,4.25 | smd 1.2 x 0.3: 13 4.25,-2.75; 14 4.25,-2.25; 15 4.25,-1.75; 16 4.25,-1.25; 17 4.25,-0.75; 18 4.25,-0.25; 19 4.25,0.25; 20 4.25,0.75; 21 4.25,1.25; 22 4.25,1.75; 23 4.25,2.25; 24 4.25,2.75; 37 -4.25,2.75; 38 -4.25,2.25; 39 -4.25,1.75; 40 -4.25,1.25; 41 -4.25,0.75; 42 -4.25,0.25; 43 -4.25,-0.25; 44 -4.25,-0.75; 45 -4.25,-1.25; 46 -4.25,-1.75; 47 -4.25,-2.25; 48 -4.25,-2.75
SOT223 = smd 1.219 x 2.235: 1 -2.311,-3.099; 2 0,-3.099; 3 2.311,-3.099 | smd 3.6 x 2.2: 4 0,3.099
U.FL = smd 2.2 x 0.85: P$1 0,1.375; P$2 0,-1.375 | smd 1.05 x 1: P$3 1.525,0; P$4 -1.525,0
2X5 = drill 0.8 pad 1.422: 1 -4,-1; 2 -4,1; 3 -2,-1; 4 -2,1; 5 0,-1; 6 0,1; 7 2,-1; 8 2,1; 9 4,-1; 10 4,1
1X05-S = drill 1.016 square: 1 -5.08,0 | drill 1.016 octagon: 2 -2.54,0; 3 0,0; 4 2.54,0; 5 5.08,0
PH005-1-6 = drill 0.7 pad 1.016: 1 0,0; 2 1.27,0; 3 2.54,0; 4 3.81,0; 5 5.08,0; 6 6.35,0
PH005-1-2 = drill 0.7 pad 1.016: 1 0,0; 2 1.27,0
USB-MINIB = smd 2.5 x 0.5: D+ 2.5,0; D- 2.5,0.8; GND 2.5,-1.6; ID 2.5,-0.8; VBUS 2.5,1.6 | smd 2.5 x 2: MTN1 -3,4.5; MTN2 2.5,4.5; MTN3 -3,-4.5; MTN4 2.5,-4.5 | hole 0.9: 0,2.2; 0,-2.2
L0402 = smd 0.5 x 0.5: 1 -0.508,0; 2 0.508,0
R0805 = smd 1.2 x 1.3: 1 -1.016,0; 2 1.016,0
R0402 = smd 0.5 x 0.5: 1 -0.508,0; 2 0.508,0
QFN20-4X4-PAD = smd 0.5 x 0.25: 1 -1.9,1; 2 -1.9,0.5; 3 -1.9,0; 4 -1.9,-0.5; 5 -1.9,-1; 11 1.9,-1; 12 1.9,-0.5; 13 1.9,0; 14 1.9,0.5; 15 1.9,1 | smd 0.25 x 0.5: 6 -1,-1.9; 7 -0.5,-1.9; 8 0,-1.9; 9 0.5,-1.9; 10 1,-1.9; 16 1,1.9; 17 0.5,1.9; 18 0,1.9; 19 -0.5,1.9; 20 -1,1.9 | smd 2.4 x 2.4: 21 0,0 | drill 0.33 pad 0.686 square: P$1 -0.838,0.838; P$2 0.838,0.838; P$3 -0.838,-0.838; P$4 0.838,-0.838; P$5 -0.838,0; P$6 0.838,-0.025; P$7 0,-0.838; P$8 0,0.838; P$9 0,0
QFN20-4X4-NRF = smd 0.5 x 0.25: 1 -1.9,1; 2 -1.9,0.5; 3 -1.9,0; 4 -1.9,-0.5; 5 -1.9,-1; 11 1.9,-1; 12 1.9,-0.5; 13 1.9,0; 14 1.9,0.5; 15 1.9,1 | smd 0.25 x 0.5: 6 -1,-1.9; 7 -0.5,-1.9; 8 0,-1.9; 9 0.5,-1.9; 10 1,-1.9; 16 1,1.9; 17 0.5,1.9; 18 0,1.9; 19 -0.5,1.9; 20 -1,1.9
QFN40-6X6 = smd 0.95 x 0.28: 1 -3.025,2.25; 2 -3.025,1.75; 3 -3.025,1.25; 4 -3.025,0.75; 5 -3.025,0.25; 6 -3.025,-0.25; 7 -3.025,-0.75; 8 -3.025,-1.25; 9 -3.025,-1.75; 10 -3.025,-2.25; 21 3.025,-2.25; 22 3.025,-1.75; 23 3.025,-1.25; 24 3.025,-0.75; 25 3.025,-0.25; 26 3.025,0.25; 27 3.025,0.75; 28 3.025,1.25; 29 3.025,1.75; 30 3.025,2.25 | smd 0.28 x 0.95: 11 -2.25,-3.025; 12 -1.75,-3.025; 13 -1.25,-3.025; 14 -0.75,-3.025; 15 -0.25,-3.025; 16 0.25,-3.025; 17 0.75,-3.025; 18 1.25,-3.025; 19 1.75,-3.025; 20 2.25,-3.025; 31 2.25,3.025; 32 1.75,3.025; 33 1.25,3.025; 34 0.75,3.025; 35 0.25,3.025; 36 -0.25,3.025; 37 -0.75,3.025; 38 -1.25,3.025; 39 -1.75,3.025; 40 -2.25,3.025 | smd 4.2 x 4.2: P$1 0,0 | drill 0.33 pad 0.686 square: P$2 -1.778,1.778; P$3 -1.067,1.778; P$4 -0.356,1.778; P$5 0.356,1.778; P$6 1.067,1.778; P$7 1.778,1.778; P$8 -1.783,1.067; P$9 -1.072,1.067; P$10 -0.361,1.067; P$11 0.351,1.067; P$12 1.062,1.067; P$13 1.773,1.067; P$14 -1.778,0.356; P$15 -1.067,0.356; P$16 -0.356,0.356; P$17 0.356,0.356; P$18 1.067,0.356; P$19 1.778,0.356; P$20 -1.783,-0.356; P$21 -1.072,-0.356; P$22 -0.361,-0.356; P$23 0.351,-0.356; P$24 1.062,-0.356; P$25 1.773,-0.356; P$26 -1.778,-1.067; P$27 -1.067,-1.067; P$28 -0.356,-1.067; P$29 0.356,-1.067; P$30 1.067,-1.067; P$31 1.778,-1.067; P$32 -1.783,-1.778; P$33 -1.072,-1.778; P$34 -0.361,-1.778; P$35 0.351,-1.778; P$36 1.062,-1.778; P$37 1.773,-1.778
QFN16-3X3-PAD = smd 0.85 x 0.3: 1 -1.655,0.75; 2 -1.655,0.25; 3 -1.655,-0.25; 4 -1.655,-0.75; 9 1.655,-0.75; 10 1.655,-0.25; 11 1.655,0.25; 12 1.655,0.75 | smd 0.3 x 0.85: 5 -0.75,-1.655; 6 -0.25,-1.655; 7 0.25,-1.655; 8 0.75,-1.655; 13 0.75,1.655; 14 0.25,1.655; 15 -0.25,1.655; 16 -0.75,1.655 | smd 1.55 x 1.55: 17 0,0

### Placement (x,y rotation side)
C20  16.75,41.1 180 top
C50  15.55,45 180 top
C_V1  30.45,10.54 180 bottom
C_V2  18.02,10.57 180 top
CA_1  4.54,35.88 270 top
CA_2  4.54,38.28 90 top
CA_3  10.97,33.21 270 top
CA_4  6.51,41.15 180 top
CA_5  11.59,39.17 0 top
CA_6  7.87,33.37 270 top
CA_7  4.77,33.37 270 top
CA_8  5.8,33.37 270 top
CA_9  10.97,35.61 90 top
CA_10  6.83,33.37 270 top
CA_11  4.91,29.72 90 top
CA_12  6.02,29.73 90 top
CA_13  13.08,33.6 270 top
CA_14  13.87,40.26 90 top
CA_15  12.8,36.85 0 top
CA_16  7.34,30.96 270 top
CA_17  12.64,30.63 90 top
CA_18  11.56,30.66 90 top
CC122  26.48,27.41 0 top
CC_41  22.83,18.63 180 top
CC_51  25.3,18.69 0 top
CC_81  29.11,19.03 270 bottom
CC_91  28.33,25.61 270 top
CC_101  28.98,24.06 180 bottom
CC_111  26.53,26.12 180 top
CC_121  24.6,25.5 90 top
CC_123  21.5,27.49 180 top
CC_124  19.69,28.02 270 top
CC_131  23.36,25.6 90 top
CC_132  23.37,28.01 90 top
CC_141  21.65,24.94 180 top
CC_151  19.7,23.75 180 top
CC_181  19.7,21.45 180 top
CC_Y1  29.12,21.91 0 bottom
CN_3  10.93,25.24 90 top
CN_4  9.87,25.24 90 top
CN_5  10.29,26.99 0 top
CN_6  10.87,28.11 180 top
CN_71  11.05,18.63 0 top
CN_91  13.44,18.62 0 top
CN_101  11.41,23.49 0 top
CN_181  3.79,22.16 90 top
CN_191  3.77,19.71 270 top
CR_1  15.15,34.36 270 top
CS_1  14.17,26.99 180 top
CS_2  5.03,11.43 180 bottom
CY_31  20.46,36.74 180 top
CY_61  20.46,35.68 0 top
CY_71  20.46,34.64 180 top
CY_81  20.46,33.6 180 top
CY_101  20.44,30.04 180 top
CY_102  19.93,31.86 90 top
CY_131  25.24,30.05 0 top
CY_161  27.64,30.06 0 top
CY_331  28.92,40 270 top
CY_341  27.9,40 90 top
CY_351  26.89,40 270 top
CY_381  23.94,38.95 0 top
CY_401  21.64,39.92 90 top
D1  22.92,11.56 0 bottom
D2  23,8.27 0 bottom
IC1  7.84,7.36 270 top
IC2  28.35,3.39 90 bottom
J1  18.83,46.78 270 top
JP1  16.53,2.14 0 top
JP2  1.19,6.76 270 top
JP3  4.19,1.31 180 bottom
JP5  12.9,11.73 180 top
JP6  28.27,6.04 180 top
L12  16.16,43.03 270 top
LA_2  5.6,31.68 180 top
LA_3  8.91,33.37 270 top
LA_4  8.48,31 90 top
LC_121  24.61,28.01 270 top
LC_122  21.54,28.63 0 top
LC_131  21.6,26.11 0 top
LN_1  7.75,25.24 270 top
LN_2  8.82,25.24 270 top
LN_3  7.86,26.99 180 top
LY_101  21.14,31.88 90 top
LY_131  22.84,30.05 0 top
R_BYP  18.99,9.66 90 bottom
RA_1  9.94,33.37 270 top
RA_2  12.01,35.11 90 top
RC_171  19.7,22.49 180 top
RN_1  13.56,20.97 270 top
RN_161  3.83,24.6 90 top
RS_1  15.44,11.2 270 top
U$1  7.83,37.56 90 top
U$2  7.23,21.24 90 top
U$3  23.62,21.77 90 top
U$4  25.61,34.65 0 top
U$5  16.49,37.9 90 top
U$6  16.45,29.32 0 top
Y2  21.07,40.03 0 bottom
YA_1  13.08,37.19 90 bottom
YN_1  11.47,21.08 90 top

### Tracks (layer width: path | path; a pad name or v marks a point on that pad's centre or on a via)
+3V3  (via drill 0.33 pad 0.18, 0.33 pad 0.69)
  Top 0.152: CY_331.2 28.39,40.01 27.28,40.01 26.89,39.61 CY_351.2 | U$6.6 16.2,26.77 | 16.2,26.77 16.2,25.12 v15.75,24.66 | CS_1.1 15.98,26.99 16.2,26.77 | v6.2,24.66 6.23,24.63 U$2.15 5.82,22.68 5.82,21.21 | U$2.7 8.9,20.74 8.64,20.47 8.64,20.04 8.41,19.86 5.89,19.86 5.82,19.94 5.82,21.21 | 5.59,21.24 5.74,21.24 5.82,21.21
  Top 0.203: U$4.33 26.86,38.12 27.2,38.46 28.68,38.46 28.93,38.71 28.93,39.46 CY_331.2 | U$4.35 25.86,37.68 25.86,38.35 26.89,39.38 CY_351.2 | U$4.3 21.81,35.9 CY_31.1 20.98,36.78 | U$4.8 21.17,33.4 CY_81.1 21,33.63 21.01,33.63 | U$4.16 25.86,30.93 26.04,30.76 26.44,30.76 CY_161.1 | U$3.18 20.53,21.77 | 20.53,21.77 CC_181.1 | U$3.4 24.13,19.02 v24.03,19.13 | CC_141.1 23.12,23.98 U$3.14 U$3.15 20.29,23.67 CC_151.1 20.21,24.57 v19.02,25.76 | U$3.9 26.4,22.27 26.98,21.69 27.38,21.69 28.22,22.53 | 28.32,22.63 28.22,22.53 | U$3.11 27.08,23.67 28.22,22.53 | 20.53,21.77 20.48,21.77 v18.87,20.17 | CN_181.1 4.2,21.24 U$2.18 5.59,21.24 | CN_71.1 10.17,18.63 9.68,19.13 9.68,20.52 9.46,20.74 U$2.7 | U$1.19 5.25,37.06 CA_2.1 v3.51,37.77 v3.5,37.77 | 21.01,34.62 20.99,34.64 CY_71.1 21.71,33.9 U$4.7 | 21.01,35.69 21,35.68 CY_61.2 20.96,35.37 21.94,34.4 U$4.6 | 24.36,39.01 U$4.38 24.36,38.87 CY_381.2 24.34,38.95 23.37,39.93 22.48,39.93 22.45,39.95 21.91,39.42 CY_401.1 21.64,39.4 U$4.40 | 15.15,36.83 U$5.16 | IC1.9 1.19,6.11 JP2.3 1.19,7.11 IC1.7 4.34,7.11 5.02,7.79 | 5.05,11.58 5.05,10.54 4.65,10.13 | 5.05,11.58 IC1.48 | v14.2,10.82 13.69,10.34 12.29,10.34 IC1.36 11.73,10.11 11.56,10.26 7.52,10.26 5.98,8.75 | 4.65,10.13 4.62,10.11 IC1.1 | JP3.5 9.27,0.91 9.63,0.48 10.97,0.48 11.4,0.99 11.4,1.7 10.59,2.52 IC1.24 | 5.02,7.79 5.98,8.75 | v5.69,7.24 5.56,7.24 5.02,7.79 | 5.05,11.58 4.09,11.58 v3.73,11.94 | 4.65,10.13 4.65,10.08 5.98,8.75
  Top 0.406: 27.43,28.7 27.15,28.98 27.15,30.04 CY_161.1 | 29.36,26.16 29.32,26.12 CC_91.1 CC_111.1 | CC_41.1 23.82,18.71 v24.03,19.13 | v19.99,37.69 19.96,37.72 19.96,38.84 20.54,39.42 CY_401.1 | 15.15,36.83 CR_1.1 15.27,34.75 v16.36,34.75 | v18.82,11.84 arc-90 19.04,11.64 C_V2.1
  Top 0.559: 25.49,38.95 26.03,39.49 CY_351.2
  Top 0.61: CY_381.2 25.49,38.95 25.98,39.45 | 27.43,28.7 28.85,28.7 29.36,28.19 29.36,26.16 29.36,23.67 28.32,22.63 v26.44,24.56 | CY_31.1 20.9,37.44 20.07,37.69 v19.99,37.69 | 20.98,36.78 21.01,36.78 21.01,35.69 21.01,34.62 21.01,33.63
  Bottom 0.203: R_BYP.2 18.85,10.82 v14.2,10.82 | JP3.5 9.27,3.66 v5.69,7.24 | v3.73,11.94 4.01,11.94 CS_2.1
  Bottom 0.406: 16.94,20.14 16.97,20.17 v18.87,20.17 19.74,21.13 20.93,21.13 23.04,18.92 v24.03,19.13 | v16.36,34.75 19.99,34.75 | R_BYP.2 18.99,10.45 19.61,9.83 22.66,9.83 23.57,8.91 23.57,4.45 24.63,3.39 IC2.2 | R_BYP.2 16.94,12.73 16.94,14.55 | R_BYP.2 arc-90 18.8,10.87 v18.82,11.84
  Bottom 0.61: v19.02,25.76 18.06,25.76 | 18.06,25.76 16.94,24.64 16.94,24.59 | 16.94,24.59 16.94,20.14 16.94,14.55 16.92,14.53 | v3.5,37.77 3.5,25.96 4.8,24.66 v6.2,24.66 v15.75,24.66 16.87,24.66 16.94,24.59 | 18.06,25.76 19.99,27.69 19.99,34.75 v19.99,37.69 | v26.44,24.56 26.44,24.41 25.6,23.37 25.6,19.66 25.15,19.2 24.11,19.2 v24.03,19.13
+5V  (via drill 0.33 pad 0.69)
  Top 0.61: v14.02,4.6 21.61,4.6 v21.64,4.62
  Bottom 0.406: 11.28,2.39 JP1.1 | D2.A 19.37,8.27 R_BYP.1 18.98,8.64
  Bottom 0.61: 11.28,2.39 11.28,3.86 12.01,4.6 v14.02,4.6 | v21.64,4.62 21.64,7.57 D2.A
A7105_CSN  (via drill 0.33 pad 0.18, 0.33 pad 0.69)
  Top 0.203: U$1.11 8.83,40.23 v9.14,40.56 | v0.74,13.11 0.99,12.98 1.6,12.98 1.88,13.26 6.71,13.26 6.86,13.06 8.96,13.06 9.09,12.98 IC1.40
  Bottom 0.203: v9.14,40.56 9.14,42.62 7.87,43.89 1.85,43.89 0.91,42.95 0.91,15.27 0.74,15.11 v0.74,13.11
BT_KEY
  Top 0.203: JP3.6 10.54,1.47 9.88,2.13 7.37,2.13 7.09,2.41 IC1.17
BT_STATE
  Top 0.203: IC1.14 5.59,3.83 5.36,4.06 4.93,4.06 4.19,3.33 JP3.1
CC_CSN  (via drill 0.33 pad 0.18, 0.33 pad 0.69)
  Top 0.152: U$3.7 25.85,21.27 26.09,21.03 26.09,19.43 v26.8,18.72
  Top 0.203: v21.21,13.61 21.03,13.77 20.65,13.39 17.8,13.39 17.27,13.92 12.6,13.92 v12.27,13.72 | IC1.31 12.05,7.57 11.51,7.57 11.12,7.95 v10.26,7.95
  Bottom 0.203: v26.8,18.72 26.8,18.01 25.98,17.2 22.55,17.2 22.3,16.94 22.3,14.86 v21.21,13.61 | v12.27,13.72 12.37,13.51 11.66,13.11 10.29,13.11 10.29,10.92 10.49,10.74 10.49,8.15 v10.26,7.95
CYRF_CSN  (via drill 0.33 pad 0.18, 0.33 pad 0.69)
  Top 0.203: U$4.24 29.37,33.9 v29.62,33.66 | v13.08,13.31 13.26,13.49 17.07,13.49 17.6,12.95 21.59,12.95 22.45,13.82 29.49,13.82 v30.33,12.98 | v10.87,7.34 11.1,7.11 IC1.30
  Bottom 0.203: v30.33,12.98 30.33,15.21 31.22,16.1 31.22,33.07 30.63,33.66 v29.62,33.66 | v13.08,13.31 13.01,13.08 12.93,13.01 12.93,12.68 10.82,12.68 10.82,11.05 11,10.87 11,7.87 10.87,7.75 v10.87,7.34
MISO  (via drill 0.33 pad 0.18, 0.33 pad 0.69)
  Top 0.152: U$2.5 8.32,19.34 v8.89,18.52 | U$3.2 23.12,19.67 22.78,19.33 22.12,19.33 21.64,18.85 21.64,18.69
  Top 0.203: U$4.28 29.22,35.9 v29.64,36.32 | 21.64,18.69 21.57,18.69 v21.54,18.67 | U$1.16 5.93,38.64 v4.47,40.11 | v2.56,14.88 v8.38,14.88 8.59,15.14 19.07,15.14 19.56,15.06 v19.76,14.86 19.99,15.09 32.05,15.09 v32.26,14.88 | v8.38,7.06 9.7,7.06 11.15,5.61 IC1.27 12.16,5.56 17.78,5.56 18.03,5.31 20.07,5.31 v20.52,5.77
  Bottom 0.203: v29.64,36.32 30.05,36.32 32.49,33.88 32.49,15.11 v32.26,14.88 | 21.61,18.59 v21.54,18.67 19.76,16.89 v19.76,14.86 | v4.47,40.11 2.13,40.11 2.13,15.32 v2.56,14.88 | v8.89,18.52 8.38,18.01 v8.38,14.88 v8.38,7.06 | v20.52,5.77 JP1.10
MOSI  (via drill 0.33 pad 0.18, 0.33 pad 0.69)
  Top 0.152: U$2.4 7.73,18.84 v8.03,18.52 | U$3.20 20.97,20.77 v20.55,20.35 20.42,20.37
  Top 0.203: U$4.27 v29.66,35.4 v29.67,35.41 | U$1.14 7.33,40.04 7.01,40.36 5.46,40.36 v4.9,40.92 | v1.96,14.28 v7.77,14.28 8.69,14.28 9.12,14.73 18.8,14.73 v19,14.45 19.23,14.45 19.41,14.25 20.12,14.25 20.5,14.66 31.27,14.66 v31.65,14.28 | v7.77,7.72 9.63,7.72 11.23,6.12 12.08,6.12 IC1.28 12.1,6.17 18.11,6.17 v18.34,5.94
  Bottom 0.203: v29.67,35.41 30.38,35.41 32.08,33.68 32.08,15.65 31.65,15.19 v31.65,14.28 | v4.9,40.92 4.9,42.39 4.22,43.08 2.31,43.08 1.73,42.49 1.73,14.48 v1.96,14.28 | v8.03,18.52 7.77,18.26 v7.77,14.28 v7.77,7.72 | v18.34,5.94 18.34,3.33 JP1.8 | v19,14.45 19,16.92 20.68,18.59 20.68,20.58 v20.55,20.35
MUXSEL1  (via drill 0.33 pad 0.18, 0.33 pad 0.69)
  Top 0.203: U$6.7 16.7,20.97 v14.86,19.13 | v10.52,13.72 9.59,13.72 IC1.39
  Bottom 0.203: v10.52,13.72 14.86,17.93 v14.86,19.13
MUXSEL2  (via drill 0.33 pad 0.18, 0.33 pad 0.69)
  Top 0.203: U$6.8 17.2,20.23 v16,19.02 | v11.4,13.72 10.74,13.06 10.08,13.06 10.09,13.05 IC1.38
  Bottom 0.203: v11.4,13.72 16,18.14 v16,19.02
N$1
  Top 0.152: 10.55,22.24 10.6,22.24 11.73,21.11 13.03,21.11
  Top 0.203: U$2.10 10.55,22.24 YN_1.3 10.62,21.85 | RN_1.1 13.4,21.48 13.03,21.11 | 10.6,22.24 10.6,23.19 CN_101.1
N$2
  Top 0.203: RN_1.2 12.8,20.46 YN_1.1 | 9.27,21.74 U$2.9 9.48,21.74 9.6,21.61 9.6,21.54 9.68,21.46 9.68,21.36 9.98,21.06 11.24,21.06 YN_1.1 | CN_91.1 12.93,19.36 YN_1.1
N$3
  Top 0.203: U$2.19 4.29,20.74 CN_191.1
N$4
  Top 0.152: U$1.6 9.73,36.34 CA_9.1 11.49,35.1 RA_2.2
N$5
  Top 0.203: U$2.13 7.23,23.78 7.04,23.98 7.04,25.55 7.21,25.73 | 7.21,25.73 7.73,25.73 LN_1.1 LN_2.1 | 7.21,25.73 7.21,26.85 LN_3.2
N$7
  Top 0.152: L12.1 16.16,44.9 | 16.16,44.9 C50.1 | 16.16,44.9 18.83,44.9 J1.P$3
N$8
  Top 0.203: LN_3.1 CN_5.1
N$9
  Top 0.203: CN_5.2 11.38,27.57 CN_6.1 11.84,28.57 U$6.4
N$10
  Top 0.203: U$2.16 5.33,22.59 RN_161.1
N$11
  Top 0.152: RA_2.1 13.09,34.61 CA_13.1
N$12  (via drill 0.33 pad 0.18)
  Top 0.152: U$1.9 9.79,38 12.12,38 CA_14.1 14.76,39.75 v14.78,39.73
  Bottom 0.152: v14.78,39.73 14.78,39.15 YA_1.3
N$14
  Top 0.203: U$3.13 23.62,24.83 CC_131.1
N$15
  Top 0.203: U$2.12 7.73,24.71 LN_1.2
N$16
  Top 0.203: U$3.12 24.12,24.51 CC_121.1
N$17  (via drill 0.33 pad 0.18)
  Top 0.152: CA_15.1 12.29,36.6 v14.17,34.72
  Top 0.203: U$1.8 10.01,37.56 10.72,36.85 CA_15.1
  Bottom 0.152: v14.17,34.72 13.59,34.72 YA_1.1
N$18
  Top 0.203: U$1.13 7.83,40.34 CA_4.1
N$24
  Top 0.203: LC_121.1 CC_132.2 22.16,28.52 LC_122.2 22.05,27.53 CC_123.1
N$25
  Top 0.203: LA_4.1 8.48,30.15 CA_18.1 11.56,30.13 CA_17.1 12.64,30.07 U$6.1
N$26
  Top 0.203: U$1.1 6.55,35.66 CA_7.1
N$27
  Top 0.203: U$1.2 7.33,35.41 CA_8.1
N$28
  Top 0.203: U$1.3 7.83,34.88 CA_10.1
N$29
  Top 0.203: U$1.4 8.33,34.34 | 8.33,34.34 CA_6.1 | LA_3.1 8.79,33.88 8.33,34.34
N$30
  Top 0.203: U$1.5 8.83,35.62 9.96,34.49 9.96,33.89 RA_1.1 10.82,33.88 CA_3.1
N$31
  Top 0.152: U$5.10 16.74,40.58 C20.1 17.26,41.42 L12.2
N$32
  Top 0.203: U$3.5 24.8,19.7 CC_51.1
N$37
  Top 0.203: U$3.17 20.43,22.27 RC_171.1
N$38  (via drill 0.33 pad 0.18)
  Top 0.203: U$3.10 v26.81,22.77
  Bottom 0.203: v26.81,22.77 CC_Y1.3 28.47,23.21 CC_101.1
N$39  (via drill 0.33 pad 0.18)
  Top 0.203: U$3.8 26.16,21.77 26.7,21.23 v26.7,21.11
  Bottom 0.203: v26.7,21.11 26.7,20.19 27.35,19.54 CC_81.1 30.22,20.65 CC_Y1.1
N$40
  Top 0.203: CC_121.2 LC_121.2 25.88,27.5 CC122.1
N$41
  Top 0.203: LC_131.2 22.15,26.11 22.17,26.09 23.34,26.09 CC_131.2 CC_132.1
N$42
  Top 0.203: U$6.15 16.2,33.37 17.22,34.39 17.22,36.23 U$5.4
N$43
  Top 0.203: CY_341.1 27.89,39.47 27.89,39.17 27.61,38.94 27.1,38.94 26.39,38.23 26.39,37.7 U$4.34
N$44  (via drill 0.33 pad 0.18)
  Top 0.203: U$4.1 22.1,36.9 21.74,37.26 21.74,37.95 v21.72,37.97
  Bottom 0.203: v21.72,37.97 21.72,38.62 Y2.1
N$45
  Top 0.203: U$4.10 22.58,32.39 LY_101.2
N$46
  Top 0.203: U$4.11 22.34,30.6 LY_131.1 22.33,30.04 CY_101.1 21.14,30.23 LY_101.1
N$47
  Top 0.203: U$4.13 24.36,30.42 CY_131.1 LY_131.2
N$48
  Top 0.203: CA_6.2 CA_10.2 6.83,31.98 | 6.83,31.98 CA_16.1 8.47,31.52 LA_4.2 | LA_2.1 6.53,31.68 6.83,31.98
N$49
  Top 0.203: U$6.12 19.91,30.07 CY_101.2 CY_102.1
N$50
  Top 0.203: LC_122.1 19.8,28.63 CC_124.1 18.15,28.53 U$6.9
NRF_CE  (via drill 0.33 pad 0.18, 0.33 pad 0.69)
  Top 0.152: U$2.1 5.65,19.34 v4.83,18.52
  Top 0.203: v4.57,12.55 4.8,12.65 8.09,12.65 IC1.42
  Bottom 0.203: v4.57,12.55 4.8,12.72 4.8,18.49 v4.83,18.52
NRF_CSN  (via drill 0.33 pad 0.18, 0.33 pad 0.69)
  Top 0.152: U$2.2 6.73,18.9 v6.35,18.49
  Top 0.203: v6.55,10.36 6.55,11.58 IC1.45
  Bottom 0.203: v6.55,10.36 6.55,18.19 v6.35,18.49
NRF_PAEN  (via drill 0.33 pad 0.18, 0.33 pad 0.69)
  Top 0.152: v9.32,23.52 8.61,23.52 U$2.11
  Top 0.203: U$2.11 8.23,24.14 LN_2.2 CN_4.1 CN_3.1 | IC1.11 6.23,5.11 6.53,5.41 6.53,7.47 8.66,9.6 v9.02,9.6
  Bottom 0.203: v9.32,23.52 9.93,22.91 9.93,15.6 9.02,14.68 v9.02,9.6
PPM  (via drill 0.33 pad 0.69)
  Top 0.203: IC1.10 2.31,5.61 v2.08,5.38
  Bottom 0.203: JP2.1 2.56,11.84 2.56,5.87 v2.08,5.38
RF_CSN
  Top 0.203: IC1.25 12.09,3.58 JP1.2
RX_EN  (via drill 0.33 pad 0.18, 0.33 pad 0.69)
  Top 0.203: U$5.6 18.64,37.65 19.05,37.24 19.05,36.52 18.39,35.87 18.39,32.64 v18.36,32.61 | v14.78,25.81 v14.78,23.34 | v9.88,4.45 9.59,4.3 IC1.22
  Bottom 0.203: v18.36,32.61 16.15,32.61 14.48,30.94 14.48,26.11 v14.78,25.81 | v14.78,23.34 13.95,22.66 13.44,22.66 10.77,20.02 10.77,15.21 9.88,14.33 9.88,10.67 10.06,10.52 10.06,8.64 9.53,8.13 9.53,5.54 9.88,5.18 v9.88,4.45
SCK  (via drill 0.33 pad 0.18, 0.33 pad 0.69)
  Top 0.152: U$2.3 7.23,18.51 v7.19,18.49 | U$3.1 21.62,19.87 21.49,19.74 20.02,19.74 v19.76,19.99
  Top 0.203: U$4.25 29.47,34.4 v29.64,34.57 | U$1.12 8.33,41.07 v8.41,41.15 | v1.37,13.66 v7.16,13.66 8.84,13.66 9.32,14.33 17.73,14.33 v18.21,14.05 18.52,14.05 18.69,13.87 18.72,13.87 18.8,13.79 20.32,13.79 20.78,14.25 30.45,14.25 v31.04,13.66 | v7.42,6.93 7.62,6.93 8.13,6.43 9.75,6.43 11.07,5.11 IC1.26 13.13,5.11 13.13,4.47 14.46,3.14 JP1.4
  Bottom 0.152: v19.76,19.99 18.21,18.44 v18.21,14.05
  Bottom 0.203: v8.41,41.15 8.74,41.48 8.74,42.37 7.62,43.48 2.06,43.48 1.32,42.75 1.32,13.72 v1.37,13.66 | v31.04,13.66 31.04,15.19 31.62,15.82 31.62,33.43 30.48,34.57 v29.64,34.57 | v7.42,6.93 7.16,7.16 v7.16,13.66 7.16,18.47 v7.19,18.49
SWCLK
  Top 0.203: IC1.37 10.71,11.73 JP5.2
SWDIO  (via drill 0.33 pad 0.69)
  Top 0.203: 12.07,9.09 IC1.34 12.11,9.09 13.31,9.09 v13.49,9.27
  Bottom 0.203: JP5.1 12.9,9.68 v13.49,9.27
TX_EN  (via drill 0.33 pad 0.18, 0.33 pad 0.69)
  Top 0.203: U$5.5 18.14,36.46 17.93,36.25 17.93,33.96 v17.25,33.27 | v13.49,25.83 v13.46,23.37 | 9.07,3.13 IC1.21 v9.09,5.05
  Bottom 0.203: v17.25,33.27 15.62,33.27 13.49,31.17 v13.49,25.83 | v13.46,23.37 10.34,20.24 10.34,15.39 9.45,14.5 9.45,10.44 9.65,10.24 9.65,8.89 9.09,8.33 v9.09,5.05
UART_RX
  Top 0.203: IC1.13 5.09,2.16 6.73,2.16 JP3.3
UART_TX
  Top 0.203: IC1.12 3.38,4.4 3.38,0.89 3.79,0.48 4.98,0.48 5.46,0.97 JP3.2
UC_CSN  (via drill 0.33 pad 0.69)
  Top 0.203: IC1.29 18.84,6.61 19.3,6.15 v19.3,5.97
  Bottom 0.203: v19.3,5.97 19.56,5.71 19.56,2.08 20.5,1.14 JP1.9
USB_D+
  Top 0.203: IC1.33 23.8,8.61 23.8,7.62 23.8,7.16 23.8,6.04 24.52,6.04 JP6.D+
USB_D-
  Top 0.203: IC1.32 23.24,8.1 23.24,5.23 23.91,5.24 JP6.D-
VBUS  (via drill 0.33 pad 0.69)
  Top 0.203: v22.5,11.68 22.5,11.99 22.02,12.47 17.4,12.47 16.97,12.9 16,12.9 15.98,12.93 15.45,12.4 RS_1.1 14.12,11.71 13.18,10.77 11.38,10.77 11.28,10.67 7.59,10.67 IC1.43 | 7.57,11.59 IC1.43 | IC1.43 IC1.44
  Top 0.406: JP6.VBUS 25.79,4.42 27.38,4.42 28.47,5.51 29.13,5.51 29.72,6.33 29.72,8.33 28.7,9.3 27.96,9.3 26.67,8.61 24.56,8.61 23.47,9.7 23.47,9.73 22.5,10.69 v22.5,11.68
  Bottom 0.406: v22.5,11.68 20.99,11.68 D1.A
VIN_LDO
  Bottom 0.406: C_V1.1 27.73,10.54 26.72,11.56 D1.C 25.05,11.49 D2.C 25.26,8.06 IC2.3
VPLL_7105  (via drill 0.33 pad 0.18)
  Top 0.152: U$1.20 5.93,36.34 v5.44,35.84 | 9.77,38.53 10.44,38.53 CA_5.1
  Top 0.203: U$1.20 4.71,36.56 CA_1.1 | 9.77,38.53 U$1.10 9.73,39.59 v9.7,39.62 | CA_11.1 6.01,29.21 CA_12.1 9.92,29.22 v9.93,29.21 | LA_3.2 RA_1.2 v9.93,31.27
  Bottom 0.152: v5.44,35.84 5.44,35.51 5.61,35.33 9.93,35.33 9.93,35.89
  Bottom 0.203: v9.7,39.62 9.93,39.62 9.93,35.89 v9.93,31.27 v9.93,29.21
VSS  (via drill 0.33 pad 0.69)
  Top 0.152: 6,42.99 8.87,43.1 | 1.75,39.12 1.7,39.06 | 1.73,29.61 1.7,29.64 | 8.87,43.1 | U$6.17 16.2,29.57 U$6.2 U$6.3 14.74,29.01 11.25,29.01 CN_6.2 | 15.61,37.65 U$5.15 13.82,37.64 13.31,37.13 CA_15.2 | 15.61,37.65 16.23,37.03 16.23,36.25 U$5.2 | 15.61,37.65 15.74,37.77 U$5.12 U$5.11 | U$5.11 C20.2 14.24,43.1 | U$5.11 16.24,38.95 16.46,38.73 17.02,38.73 17.04,38.76 17.09,38.76 17.17,38.68 17.17,39.49 U$5.9 U$5.8 U$5.7 18.17,38.18 18.67,38.18 19.96,36.89 CY_31.2 19.95,36.73 CY_61.1 CY_71.2 CY_81.2 19.93,33.58 CY_102.2 | U$5.3 U$5.2 | U$5.2 U$5.1 | 11.56,32.71 12.44,32.71 CA_13.2 14.77,33.47 CR_1.2 15.15,31.52 U$6.16 15.7,30.07 U$6.17 | 16.7,29.57 U$6.14 U$6.13 | 16.7,29.57 U$6.11 U$6.10 | 16.7,29.57 U$6.17 | U$1.P$9 U$1.P$7 | U$1.P$7 8.72,37.56 9.22,37.06 | 9.22,37.06 U$1.7 | 9.22,37.06 6.83,37.06 U$1.15 | CA_5.2 12.27,39.17 CA_14.2 13.89,40.79 13.89,41.96 12.76,43.1 | 8.87,43.1 12.76,43.1 | 12.76,43.1 14.24,43.1 | U$6.17 15.7,28.57 U$6.5 14.34,27.66 CS_1.2 12.17,26.99 CN_3.2 | CN_3.2 CN_4.2 | CN_3.2 11.13,25.75 11.91,24.97 CN_101.2 | 1.7,19.18 1.73,19.2 CN_191.2 4.29,19.2 U$2.20 | U$2.17 4.71,21.74 CN_181.2 1.73,22.66 1.7,22.63 | RN_161.2 1.81,25.11 1.7,24.99 | CC_141.2 21.1,24.99 LC_131.1 21,26.21 CC_123.2 20.97,27.51 CC_124.2 18.29,27.51 | 19.2,23.11 CC_151.2 19.2,24.16 18.26,25.09 18.26,27.49 18.29,27.51 | 19.2,23.11 RC_171.2 CC_181.2 | 18.29,27.51 18.26,27.51 U$6.17 | 19.2,23.11 20.75,23.11 21.1,22.77 U$3.16 22.62,22.77 U$3.P$2 | U$3.P$2 U$3.P$9 | U$3.19 23.12,21.27 U$3.P$9 | CC_111.2 27.04,25.1 CC_91.2 | U$1.P$2 U$1.P$6 U$1.P$4 U$1.P$7 | U$1.P$3 U$1.P$7 | U$1.P$1 U$1.P$8 | U$3.P$2 U$3.P$8 U$3.P$1 U$3.P$5 U$3.P$3
  Top 0.152: U$3.P$9 23.65,21.8 U$3.P$6 U$3.P$4 | U$3.P$7 U$3.P$9 | U$2.14 6.73,21.77 7.26,21.23 U$2.8 | 14.24,43.1 C50.2 15.05,46.78 J1.P$2 | J1.P$1 21.59,46.78 21.59,43.12
  Top 0.203: CY_161.2 28.15,31.34 U$4.20 | CY_131.2 25.75,30.33 25.38,30.71 25.38,31.61 U$4.15 | 31.39,33.4 31.47,33.33 | U$4.21 31.45,32.4 31.47,32.38 | 31.47,32.84 31.41,32.9 U$4.22 U$4.23 | 25.81,16.83 25.88,16.76 | CC_41.2 22.34,18.71 22.35,18.69 | CA_18.2 11.56,32.71 CA_3.2 | CY_381.1 23.43,38.8 23.85,38.38 23.85,37.69 U$4.39 23.86,36.46 U$4.P$2 23.81,36.4 U$4.2 | CC_111.2 26.02,26.43 CC122.2 | v15.93,16.66 v15.92,16.66 15.92,16.74 | v29.16,16.74 28.22,16.74 28.22,16.77 | v16.56,12.01 16.56,11.02 C_V2.2 16.89,10.69 RS_1.2 14.93,10.69 14.2,9.91 13.21,9.91 12.85,9.6 IC1.35 | 8.59,4.19 8.59,4.7 8.48,4.83 8.48,5.36 8.87,5.71 9.35,5.71 9.73,5.33 9.91,5.33 10.52,4.72 10.52,4.7 | 8.59,4.19 IC1.20 | 10.52,4.7 10.52,4.22 10.08,3.79 IC1.23 | 10.52,4.7 10.82,4.7 11.2,4.32 11.2,2.87 11.91,2.16 16.5,2.16 16.53,2.13 | IC1.47 5.59,10.46 v5.69,10.36 | v5.56,16.76 4.42,16.76 4.32,16.66 | v4.82,6.61 IC1.8 | 8.59,4.19 7.24,4.19 v6.9,4.53 | U$4.4 23.44,35.4 U$4.P$14 | U$4.P$22 U$4.P$1 | U$4.36 25.36,36.53 U$4.P$4 | CA_9.2 10.87,36.12 9.93,37.06 U$1.7
  Top 0.305: U$4.31 U$4.32
  Top 0.406: CY_331.1 29,40.51 29,43.16 | CY_341.2 27.84,40.51 27.84,43.16 | CY_351.1 27,40.51 27,40.54 26.8,40.54 26.8,43.15 | 21.59,43.12 21.64,43.07 CY_401.2 | CY_161.2 31.43,30.06 31.47,30.02 | 31.25,32.4 31.47,32.18 | U$4.31 31.39,37.67 31.47,37.59 | CC_51.2 25.81,16.83 | 22.35,18.69 22.35,16.75 | CN_71.2 11.55,16.8 11.48,16.73 | CN_91.2 13.95,16.81 14.02,16.73 | 1.7,30.18 4.91,30.18 CA_11.2 CA_12.2 6.02,30.51 CA_16.2 | LA_2.2 5.1,31.65 4.77,31.65 | 4.77,31.65 1.7,31.65 | CA_8.2 5.8,32.84 5.66,32.84 5.66,32.86 CA_7.2 4.77,31.65 | CA_1.2 4.54,35.31 1.7,35.31 | CA_2.2 4.54,39.12 1.75,39.12 | CA_4.2 6,42.99 6,43.1 8.87,43.1 | CA_17.2 12.64,31.17 CA_18.2 | JP6.GND 25.78,7.64 27.33,7.64 28.32,6.66 v28.75,6.66
  Top 0.61: v17.02,9.35 17.02,10.56 C_V2.2 | JP1.5 16.53,2.13 | 16.5,2.16 16.5,3.11 JP1.6
  Top 2.54: 8.87,43.1 1.7,43.1 1.7,39.06 1.7,35.31 1.7,31.65 1.7,30.18 1.7,29.64 1.7,24.99 1.7,22.63 1.7,19.18 1.7,16.7 11.48,16.73 14.02,16.73 15.92,16.74 22.35,16.75 25.88,16.76 27.76,16.77 28.22,16.77 30.81,16.77 31.47,16.78 31.47,30.02 31.47,32.18 31.47,32.38 31.47,32.84 31.47,33.33 31.47,37.59 31.47,43.18 29,43.16 27.84,43.16
  Bottom 0.203: C_V1.2 29.16,12.85 v29.16,16.74 | 31.45,6.66 31.46,6.67 | v15.93,16.66 15.93,12.65 v16.56,12.01 | JP2.4 2.56,4.22 4.82,6.47 v4.82,6.61 | JP3.4 8,3.43 v6.9,4.53 v4.82,6.61 | v4.82,6.61 4.82,9.49 v5.69,10.36 5.69,11.28 CS_2.2 | CS_2.2 5.59,11.48 | CS_2.2 5.54,16.74 v5.56,16.76
  Bottom 0.406: IC2.1 29.14,1.08 IC2.4 31.45,6.66 29.62,6.66 v28.75,6.66 | 31.46,6.67 C_V1.2
  Bottom 0.61: JP1.6 16.53,8.86 v17.02,9.35
  pour Top: 8.69,41.91 15.52,41.91 15.52,44.3 8.64,44.3
  pour Top: 30.25,41.94 30.23,17.93 2.84,17.91 2.92,41.94 29.51,41.91
  pour Bottom: 0.51,44.27 0.56,15.57 32.61,15.6 32.74,44.37 0.48,44.27
  pour Top: 8.61,22.71 6.6,22.71 6.15,22.38 6.15,20.17 8.31,20.17 8.36,20.62 8.61,20.98
  pour Top: 28.6,41.96 16.81,41.96 16.81,44.35 28.6,44.35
